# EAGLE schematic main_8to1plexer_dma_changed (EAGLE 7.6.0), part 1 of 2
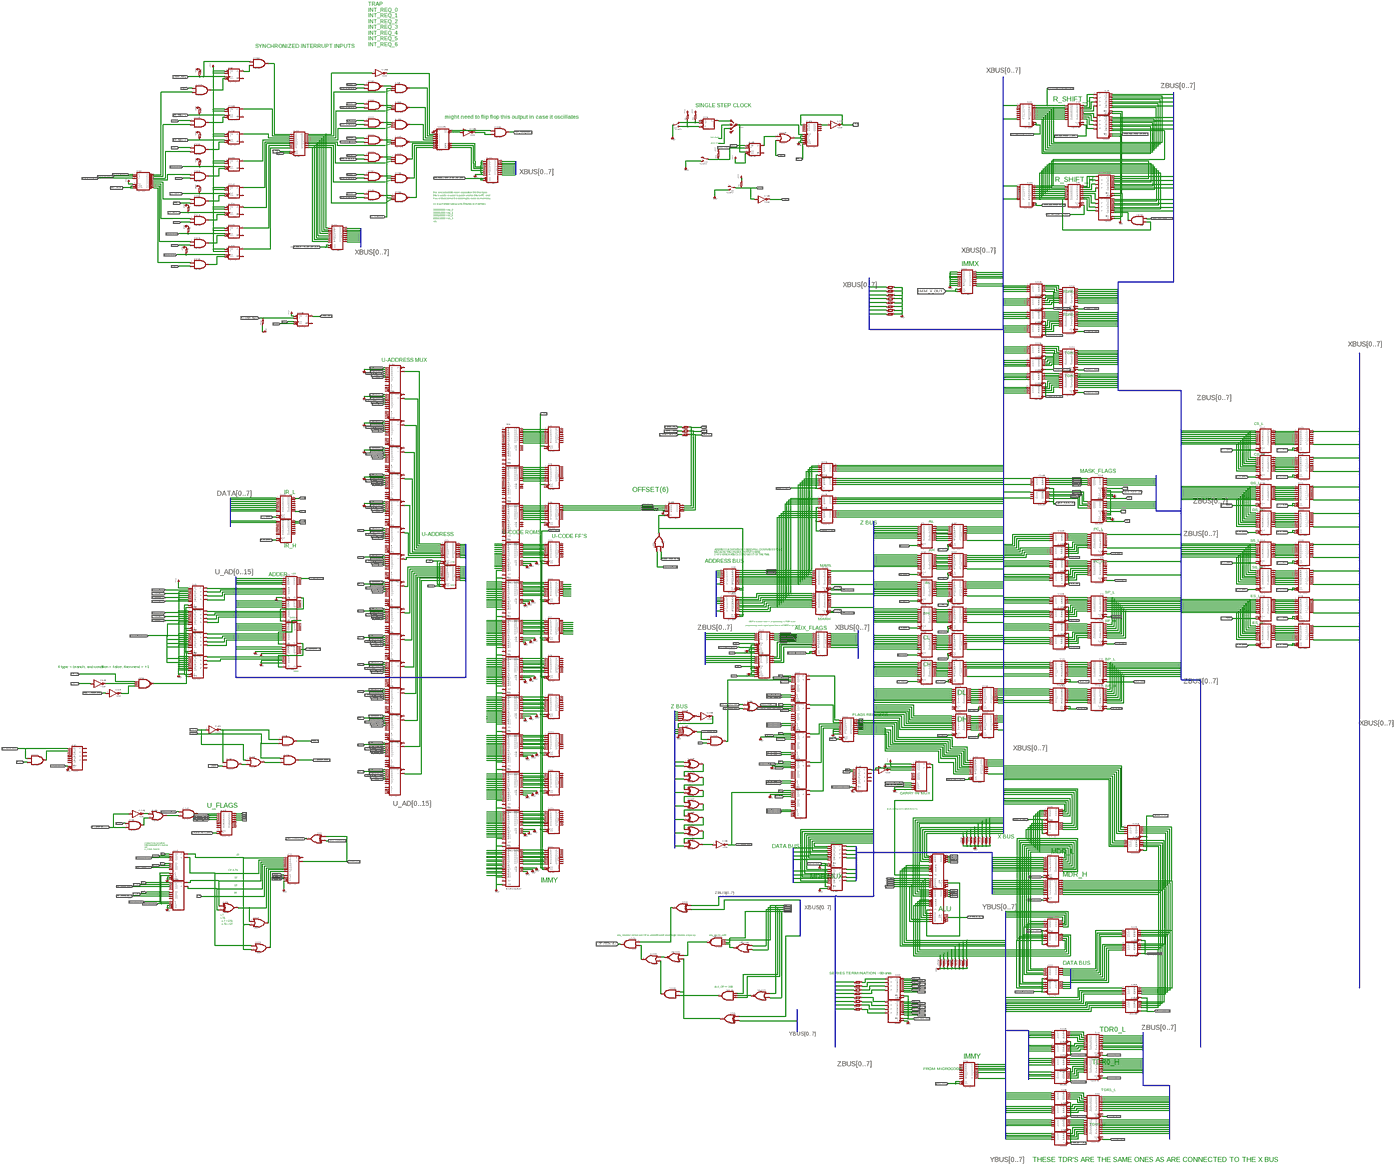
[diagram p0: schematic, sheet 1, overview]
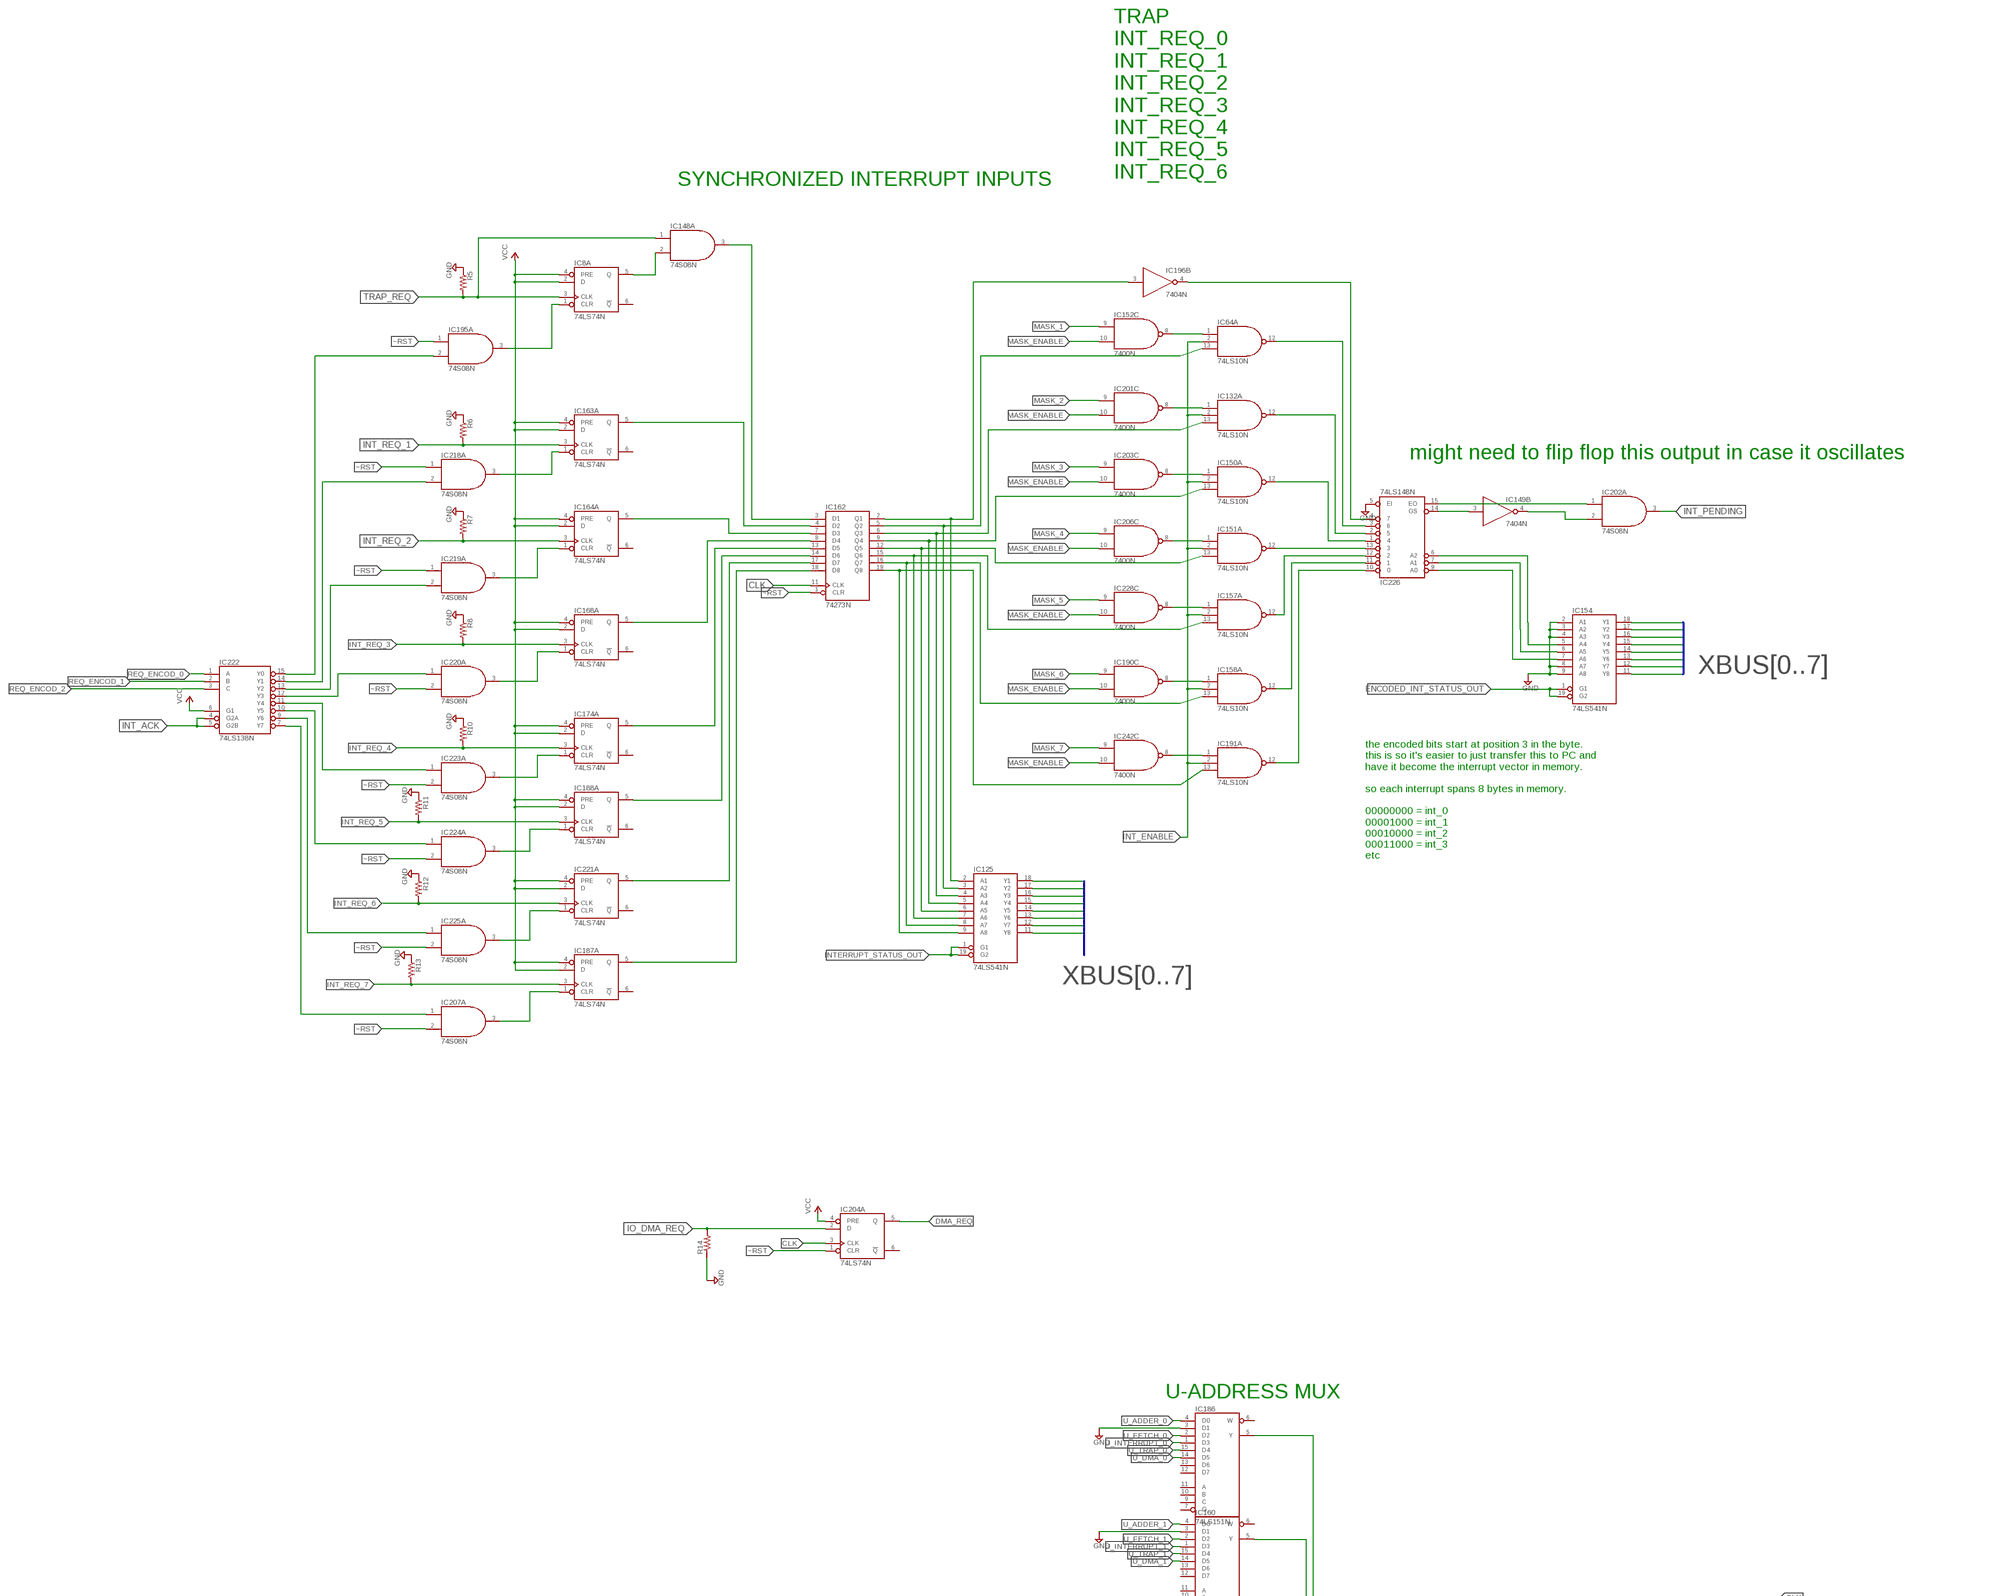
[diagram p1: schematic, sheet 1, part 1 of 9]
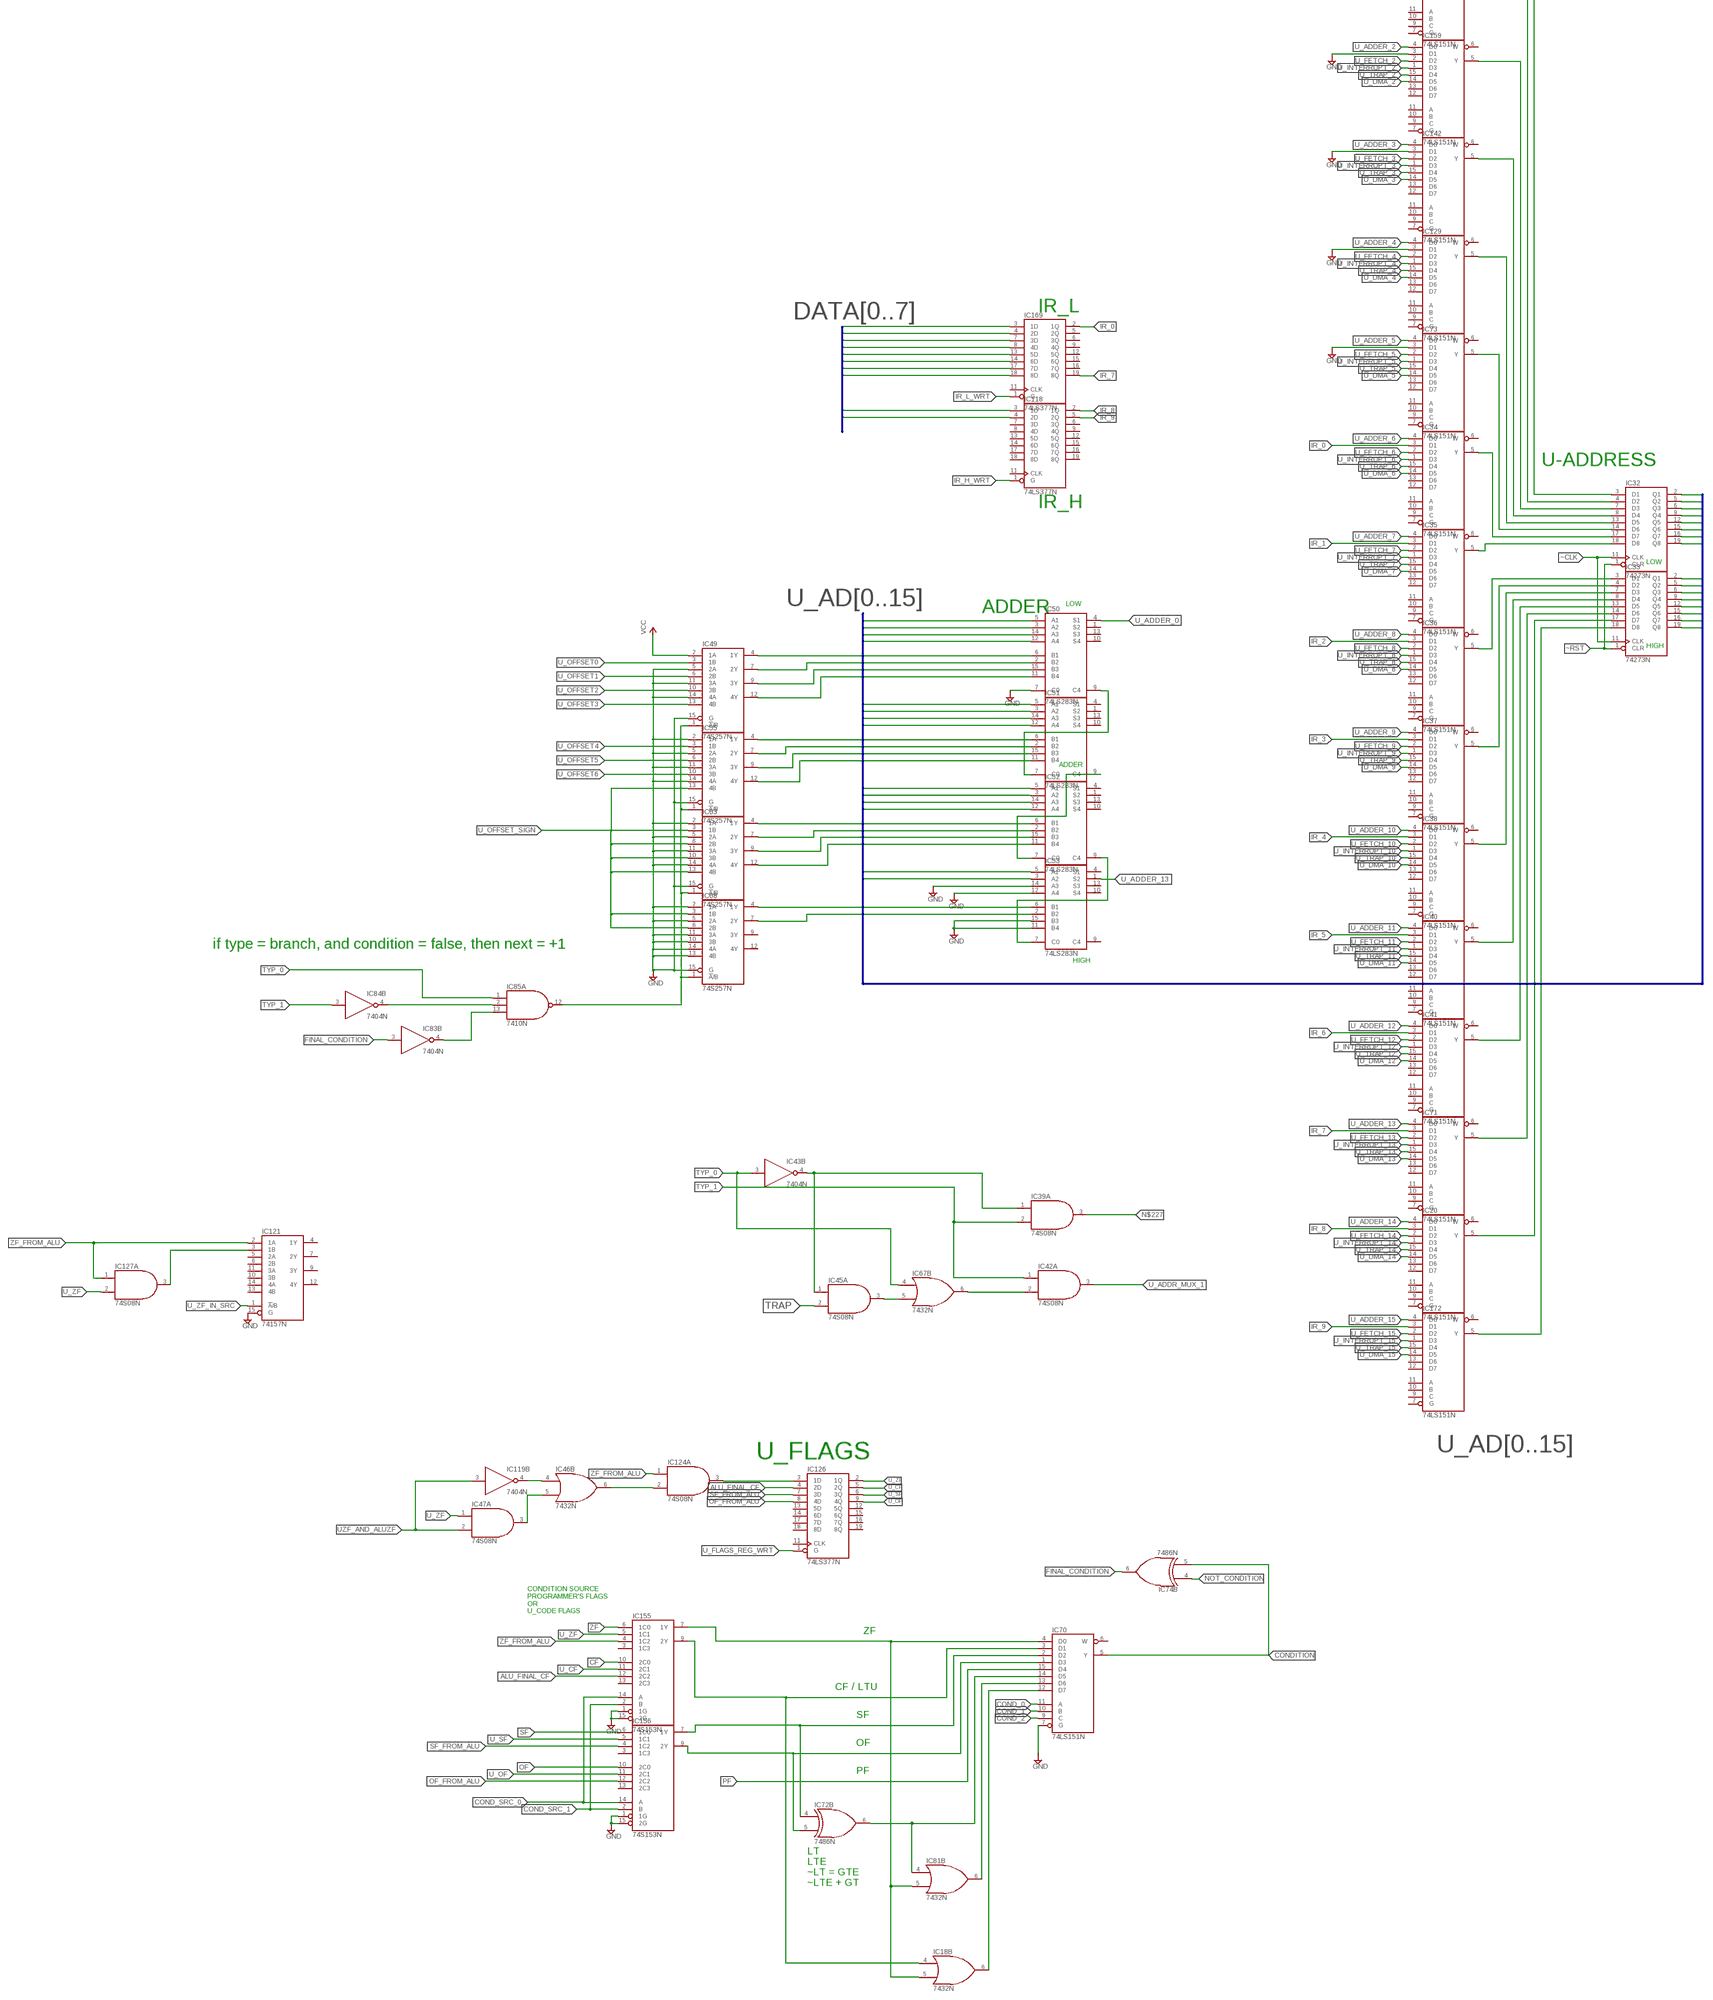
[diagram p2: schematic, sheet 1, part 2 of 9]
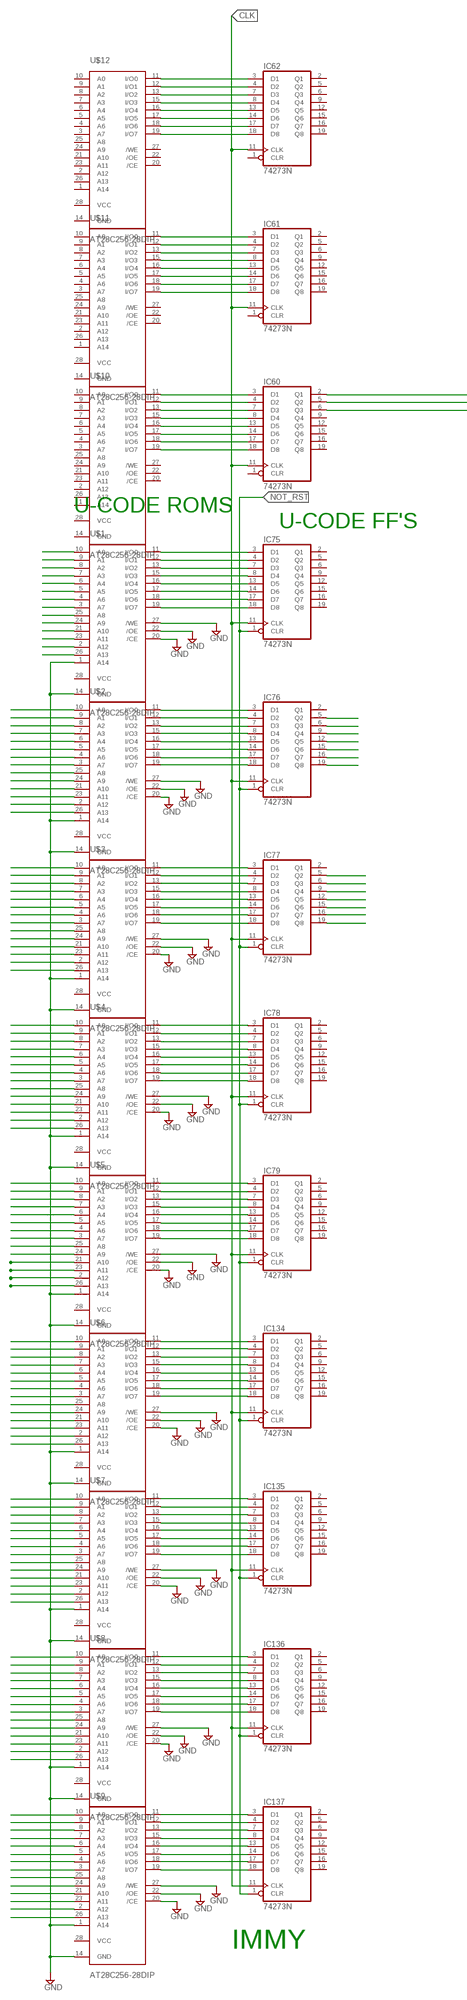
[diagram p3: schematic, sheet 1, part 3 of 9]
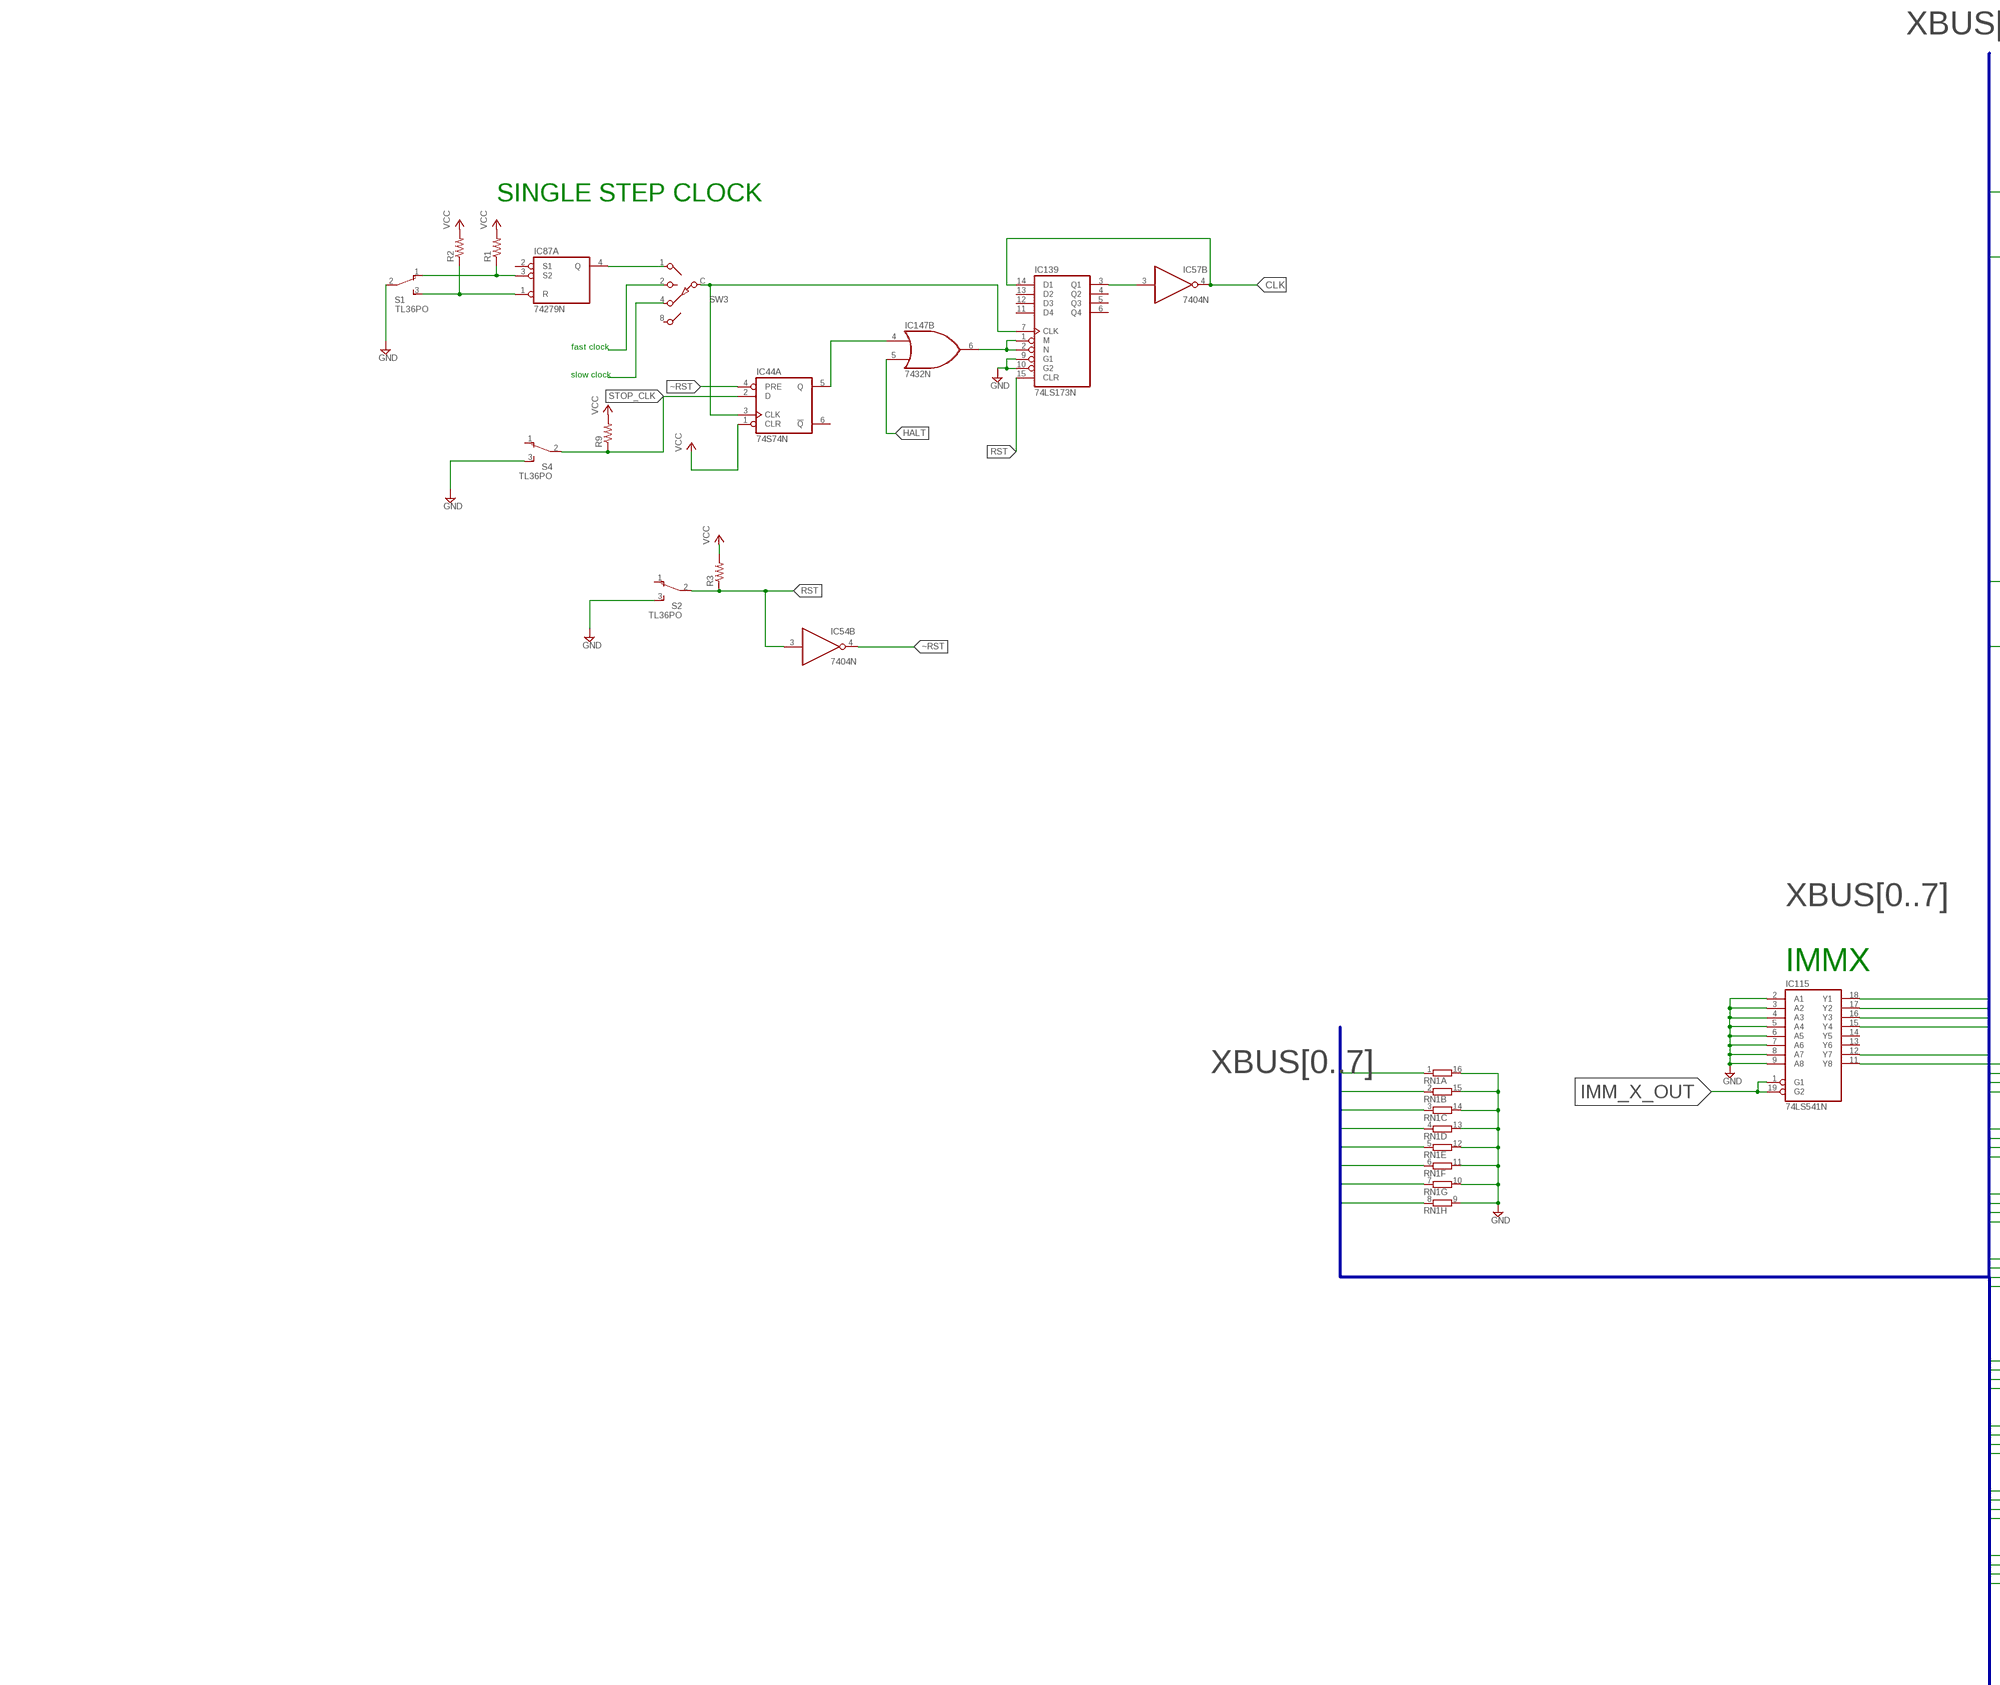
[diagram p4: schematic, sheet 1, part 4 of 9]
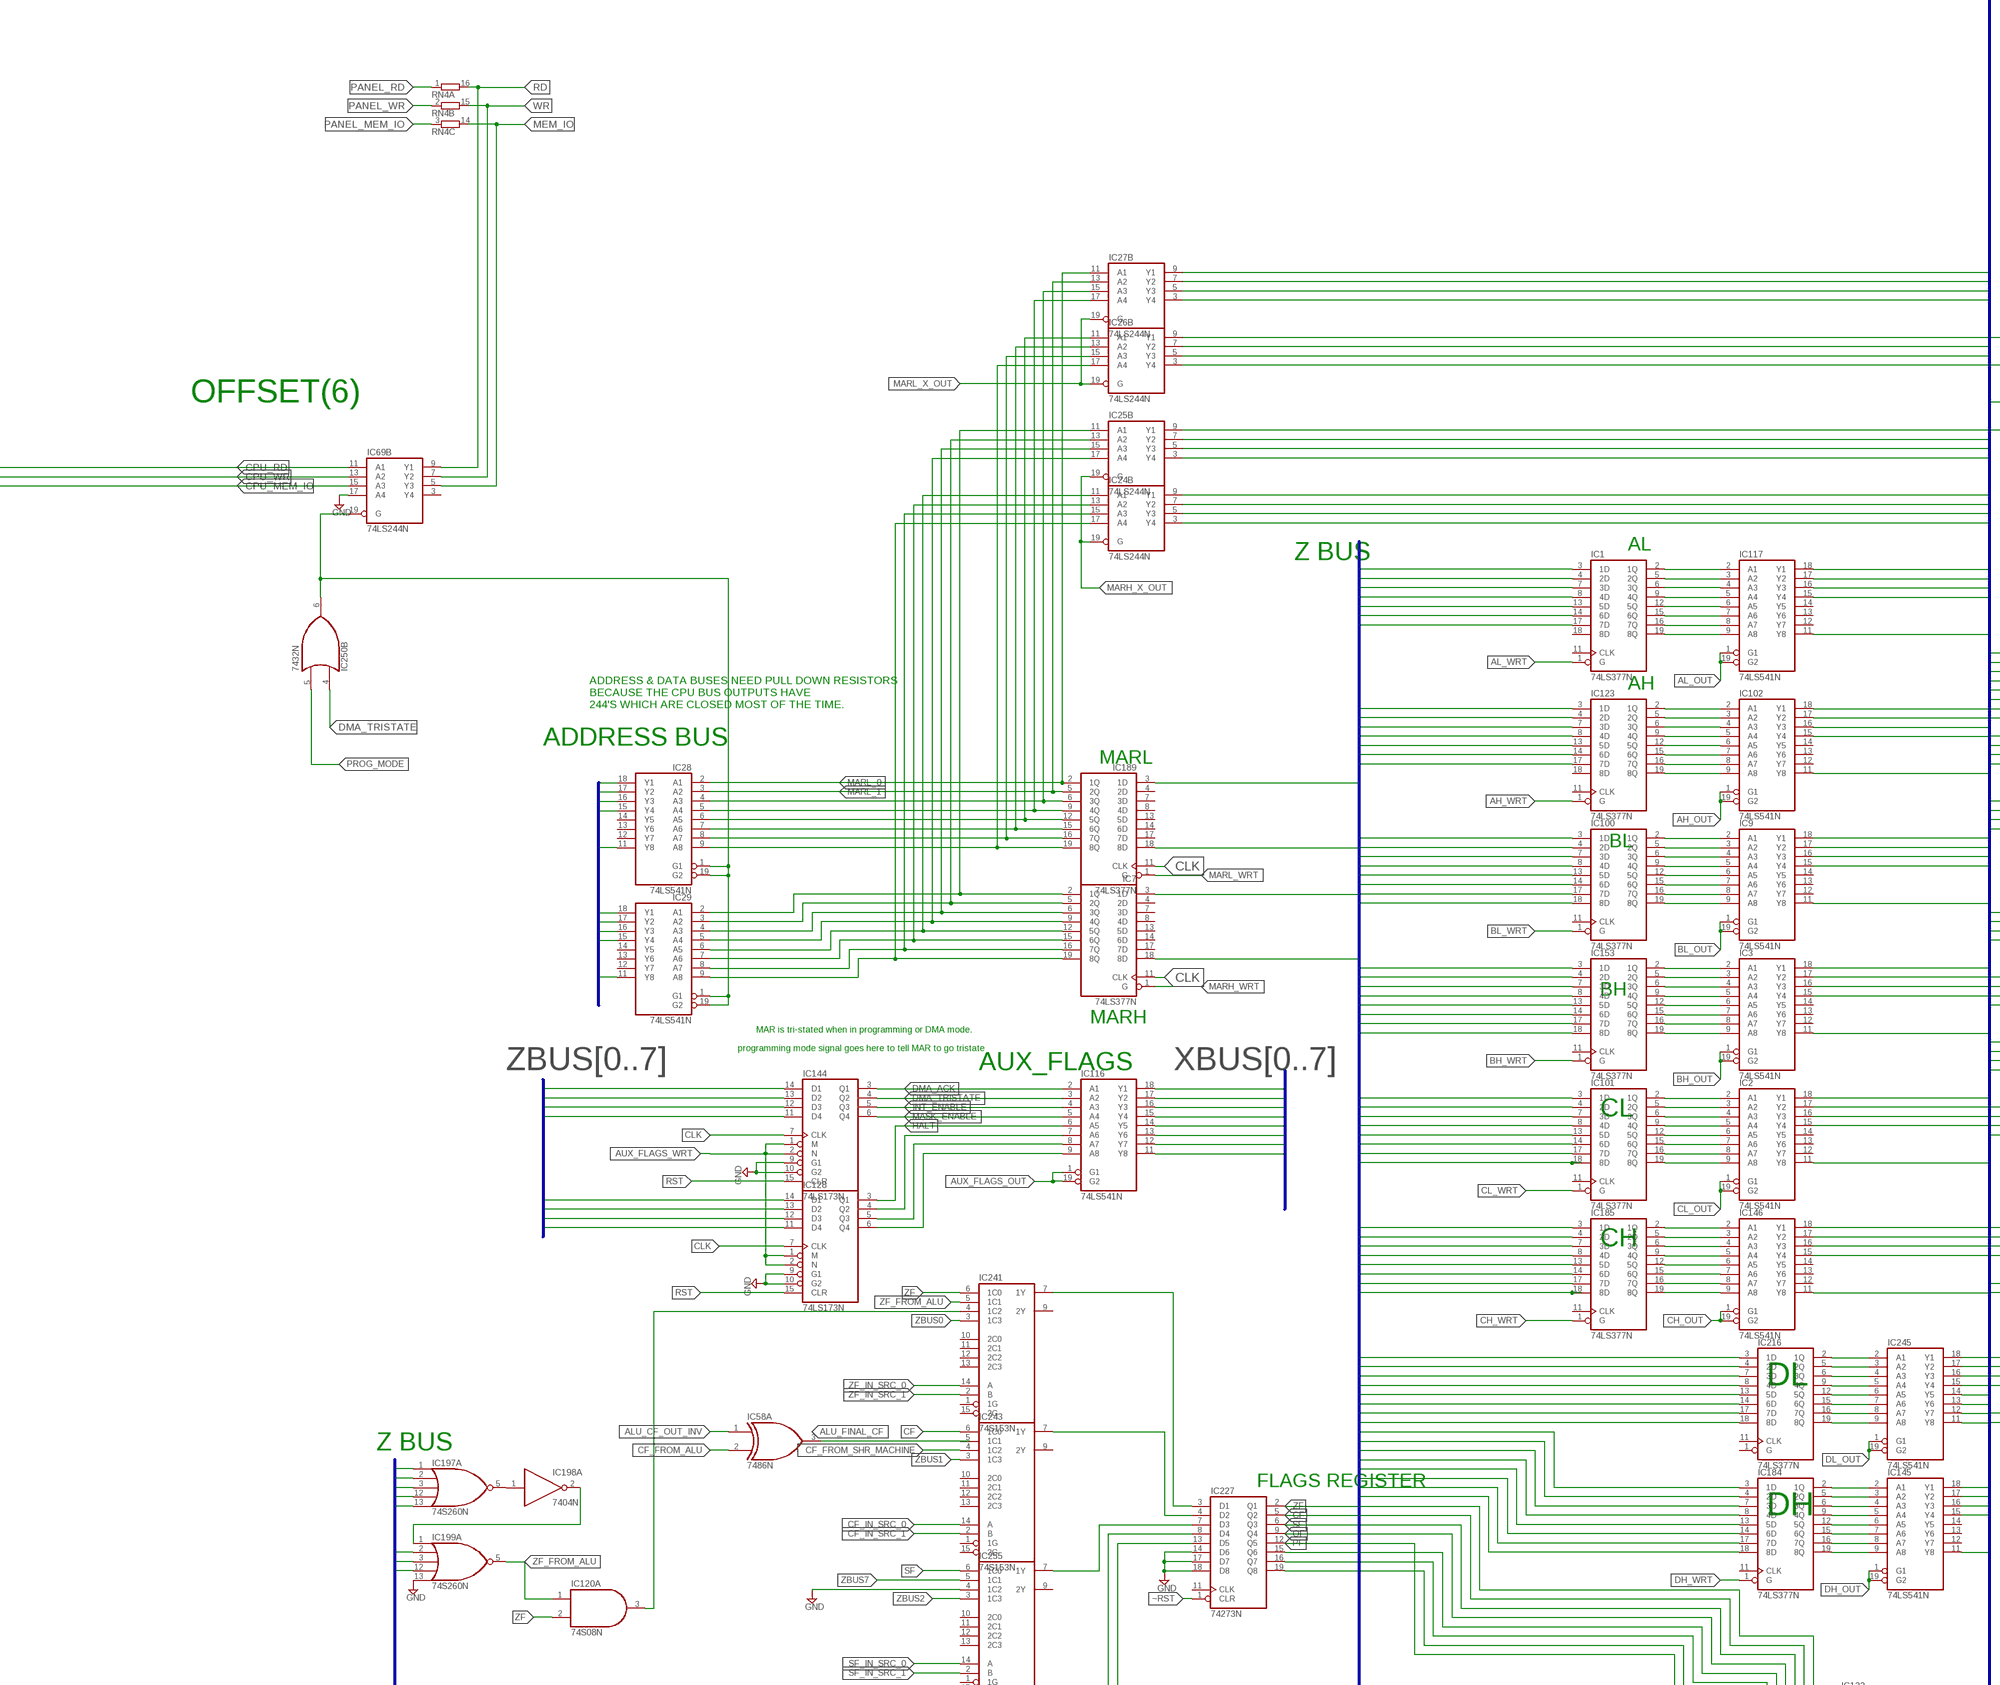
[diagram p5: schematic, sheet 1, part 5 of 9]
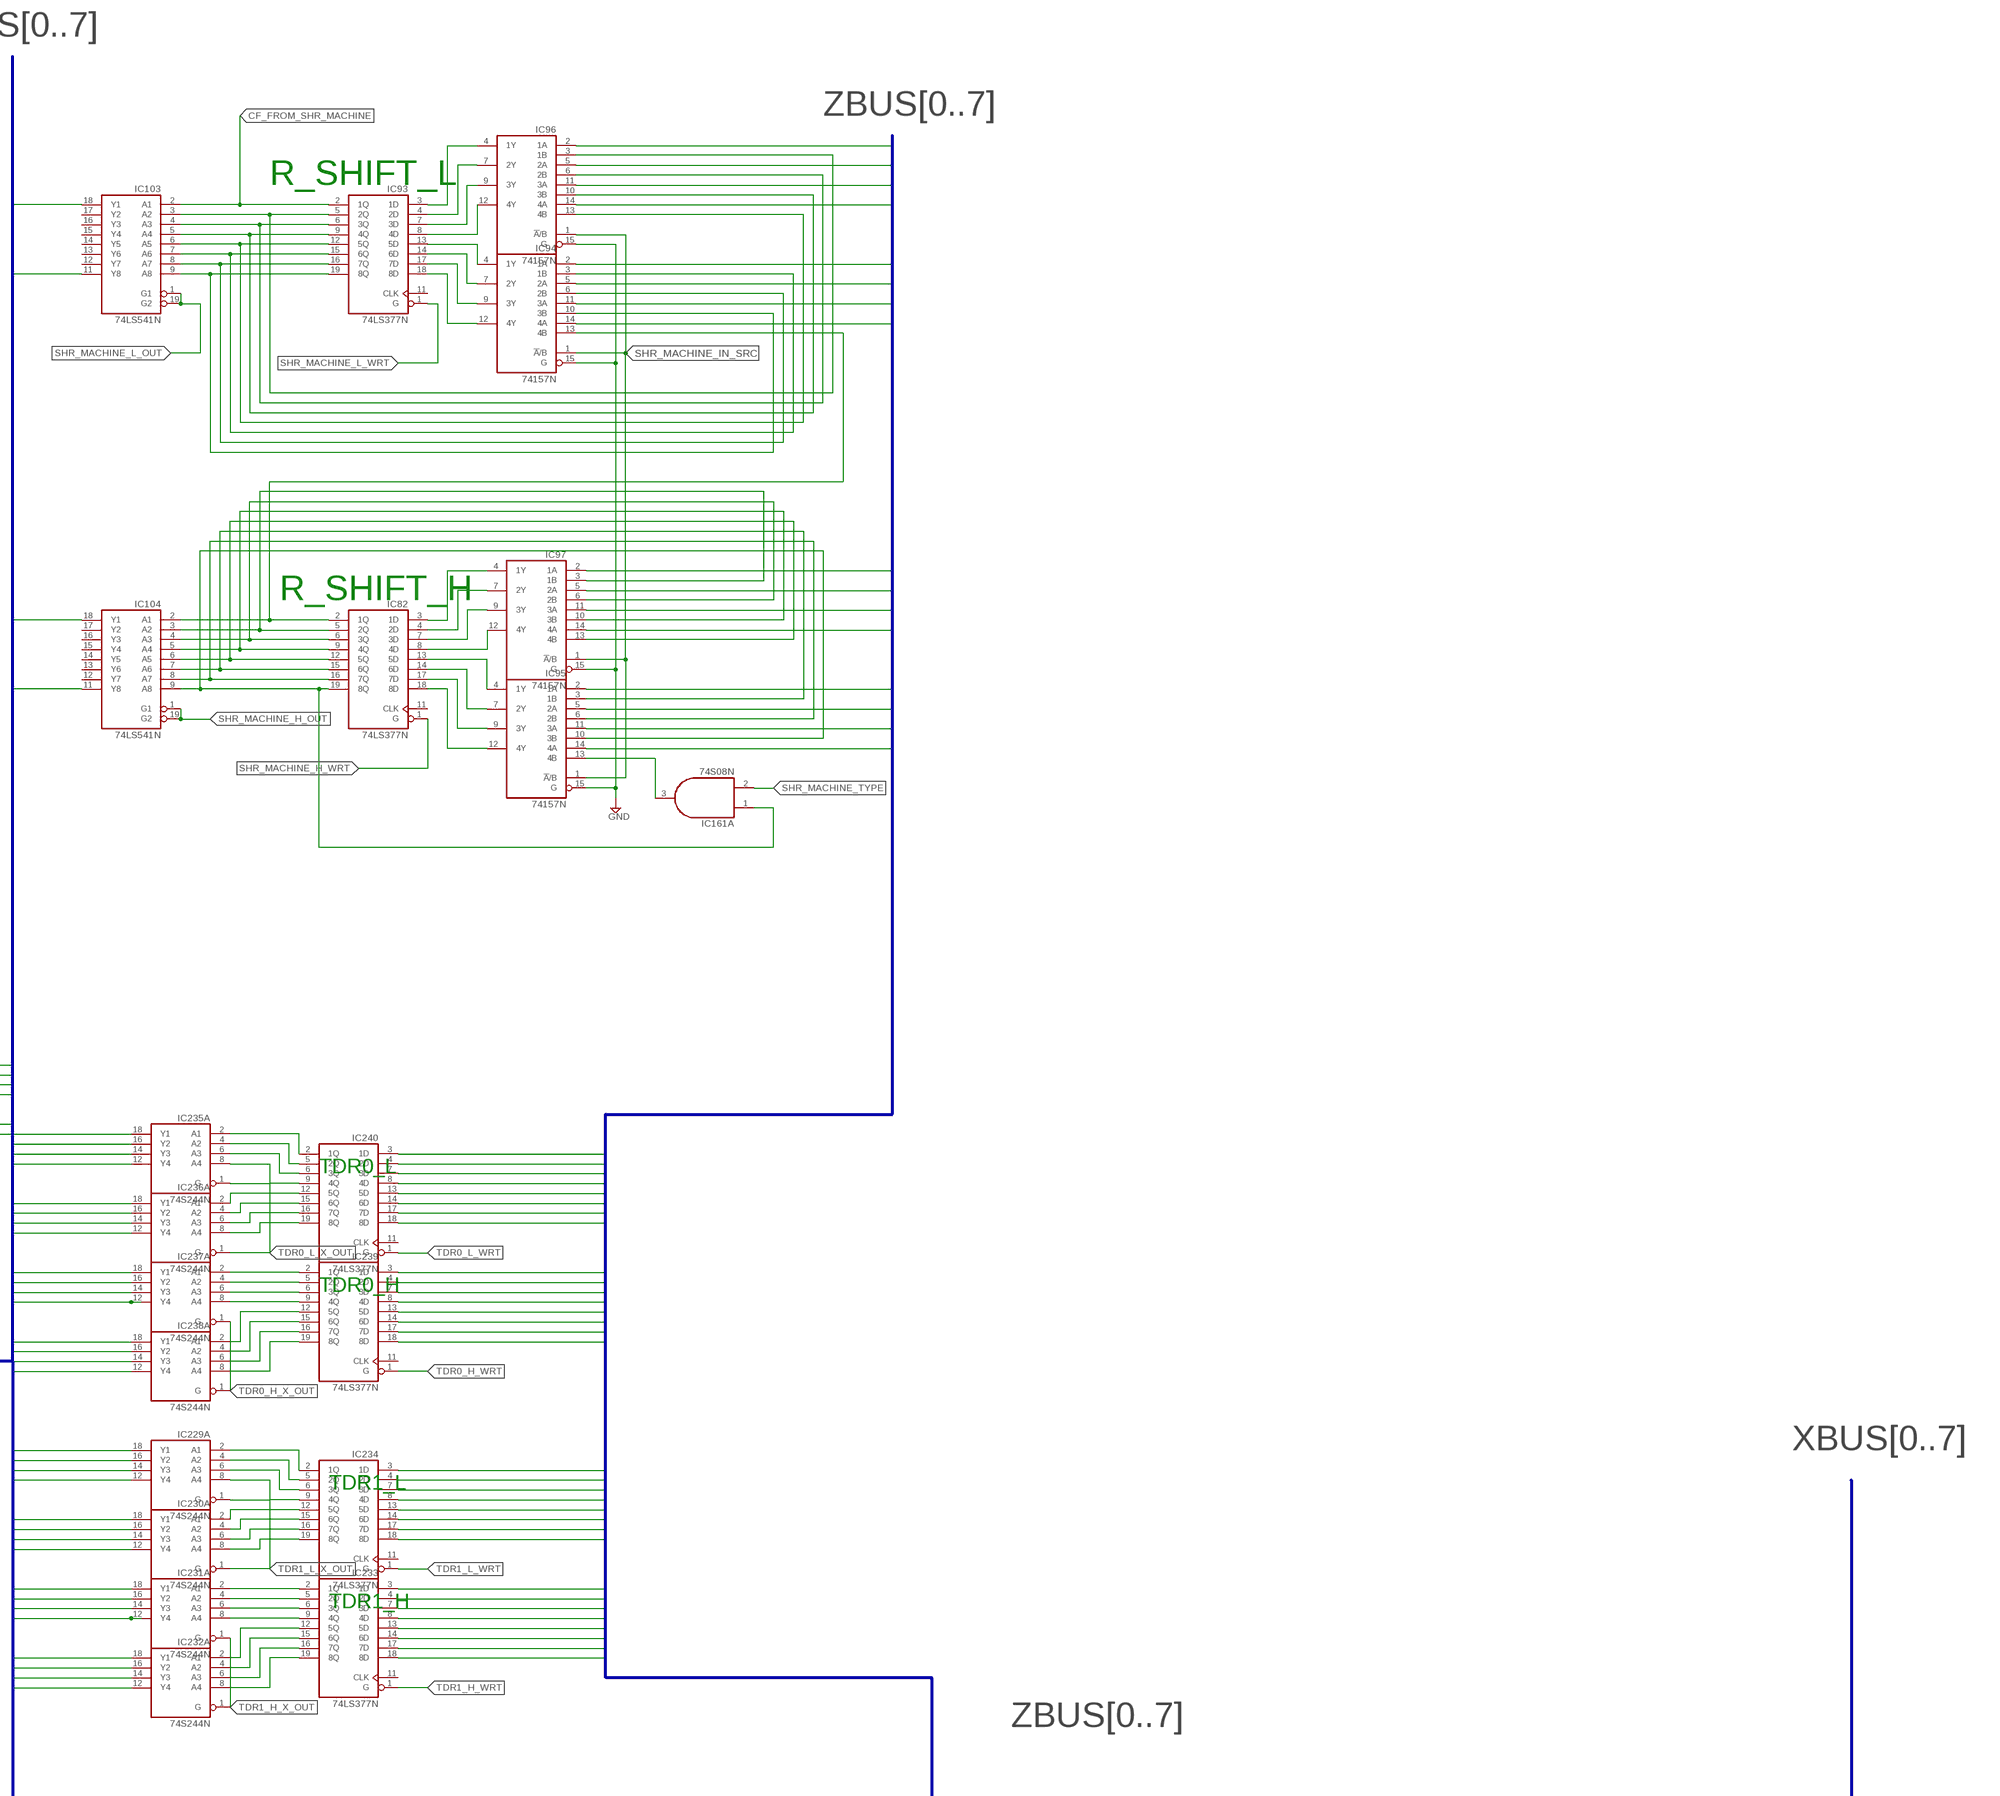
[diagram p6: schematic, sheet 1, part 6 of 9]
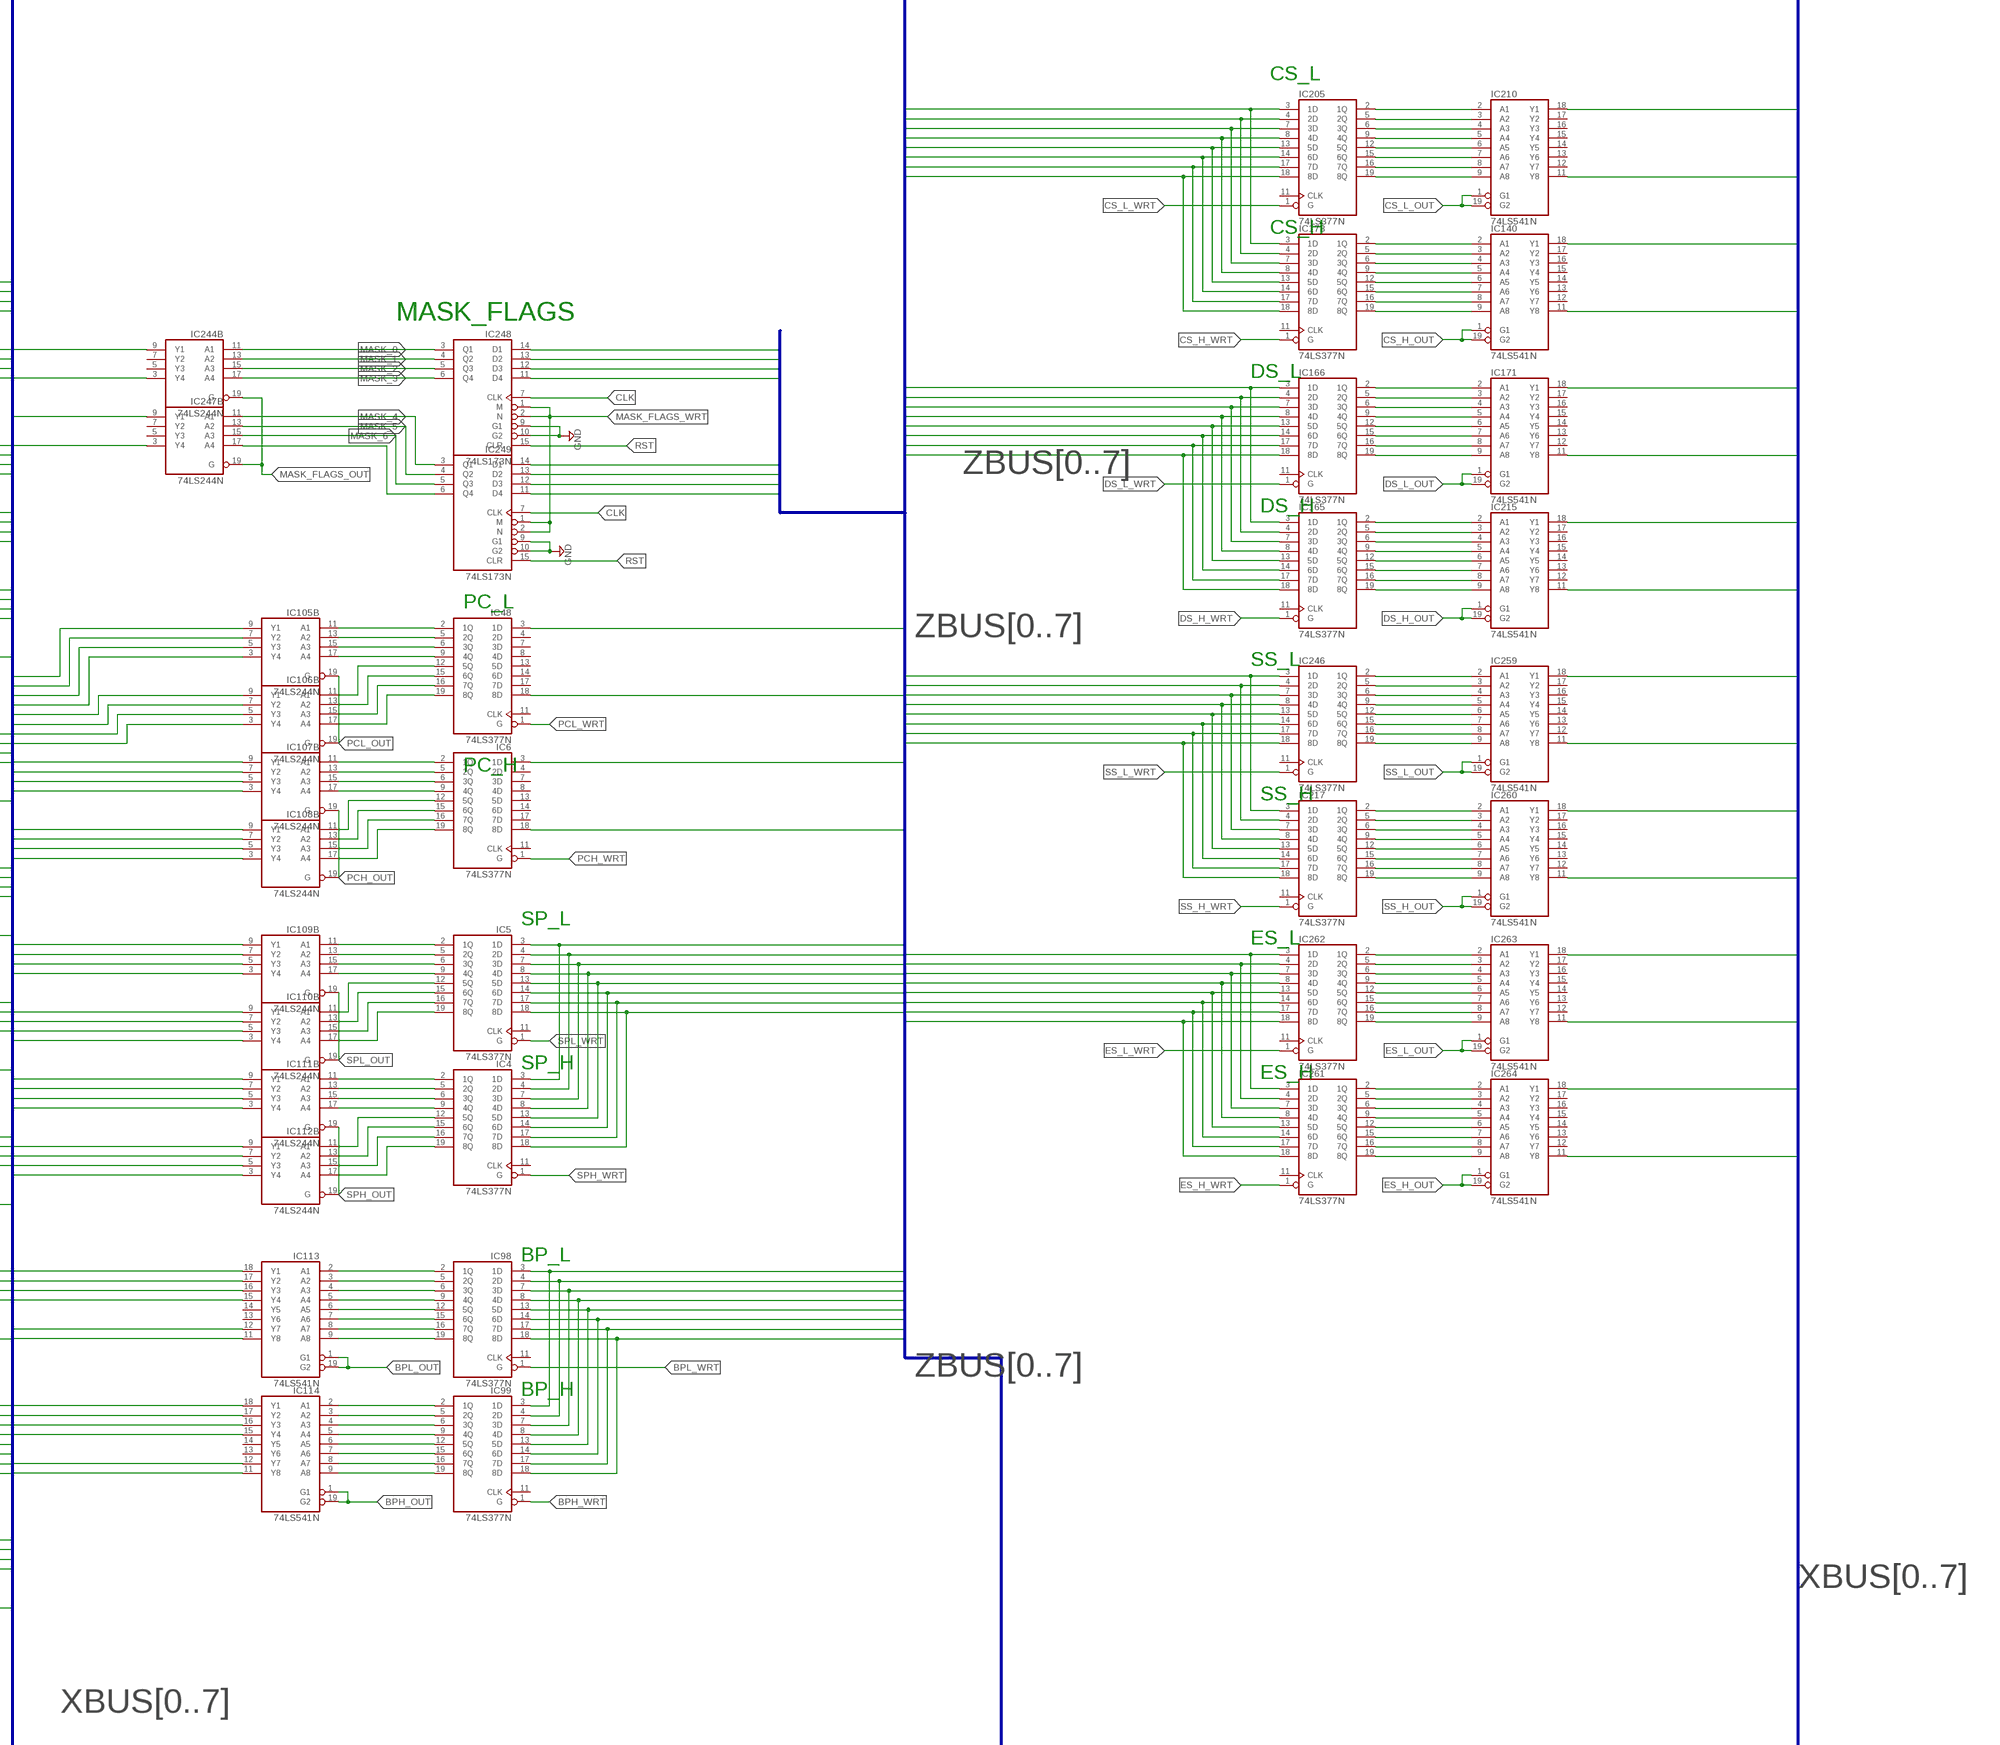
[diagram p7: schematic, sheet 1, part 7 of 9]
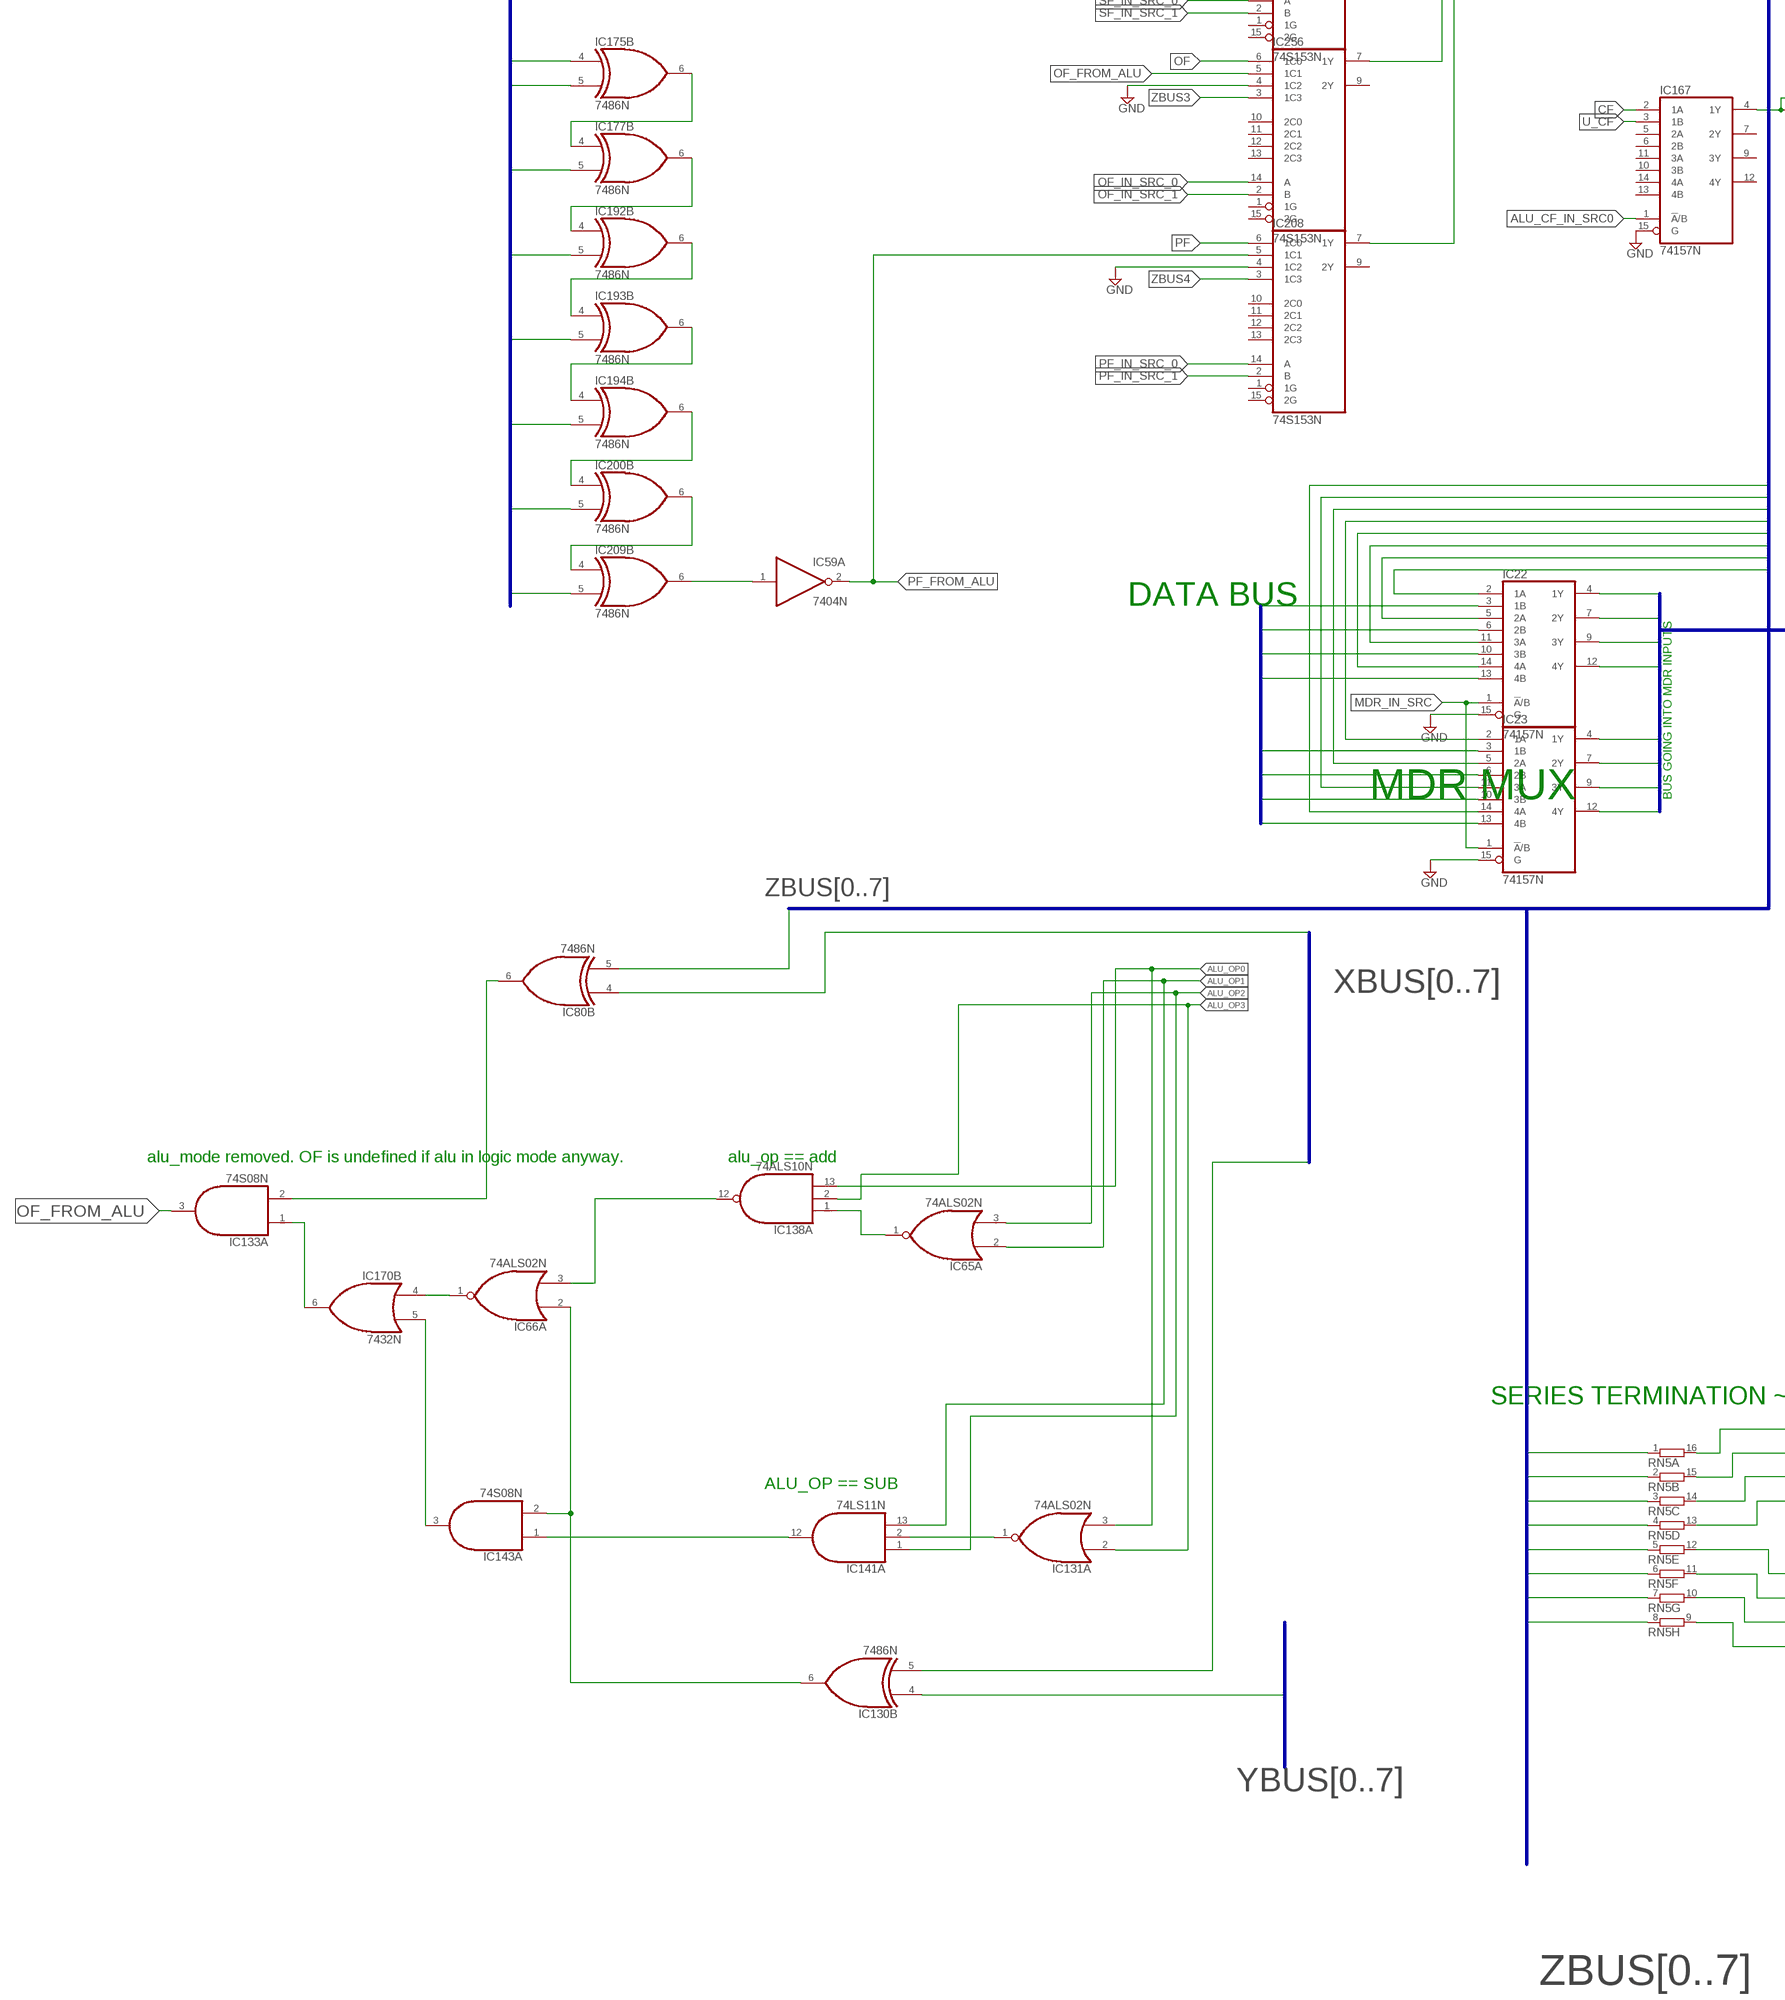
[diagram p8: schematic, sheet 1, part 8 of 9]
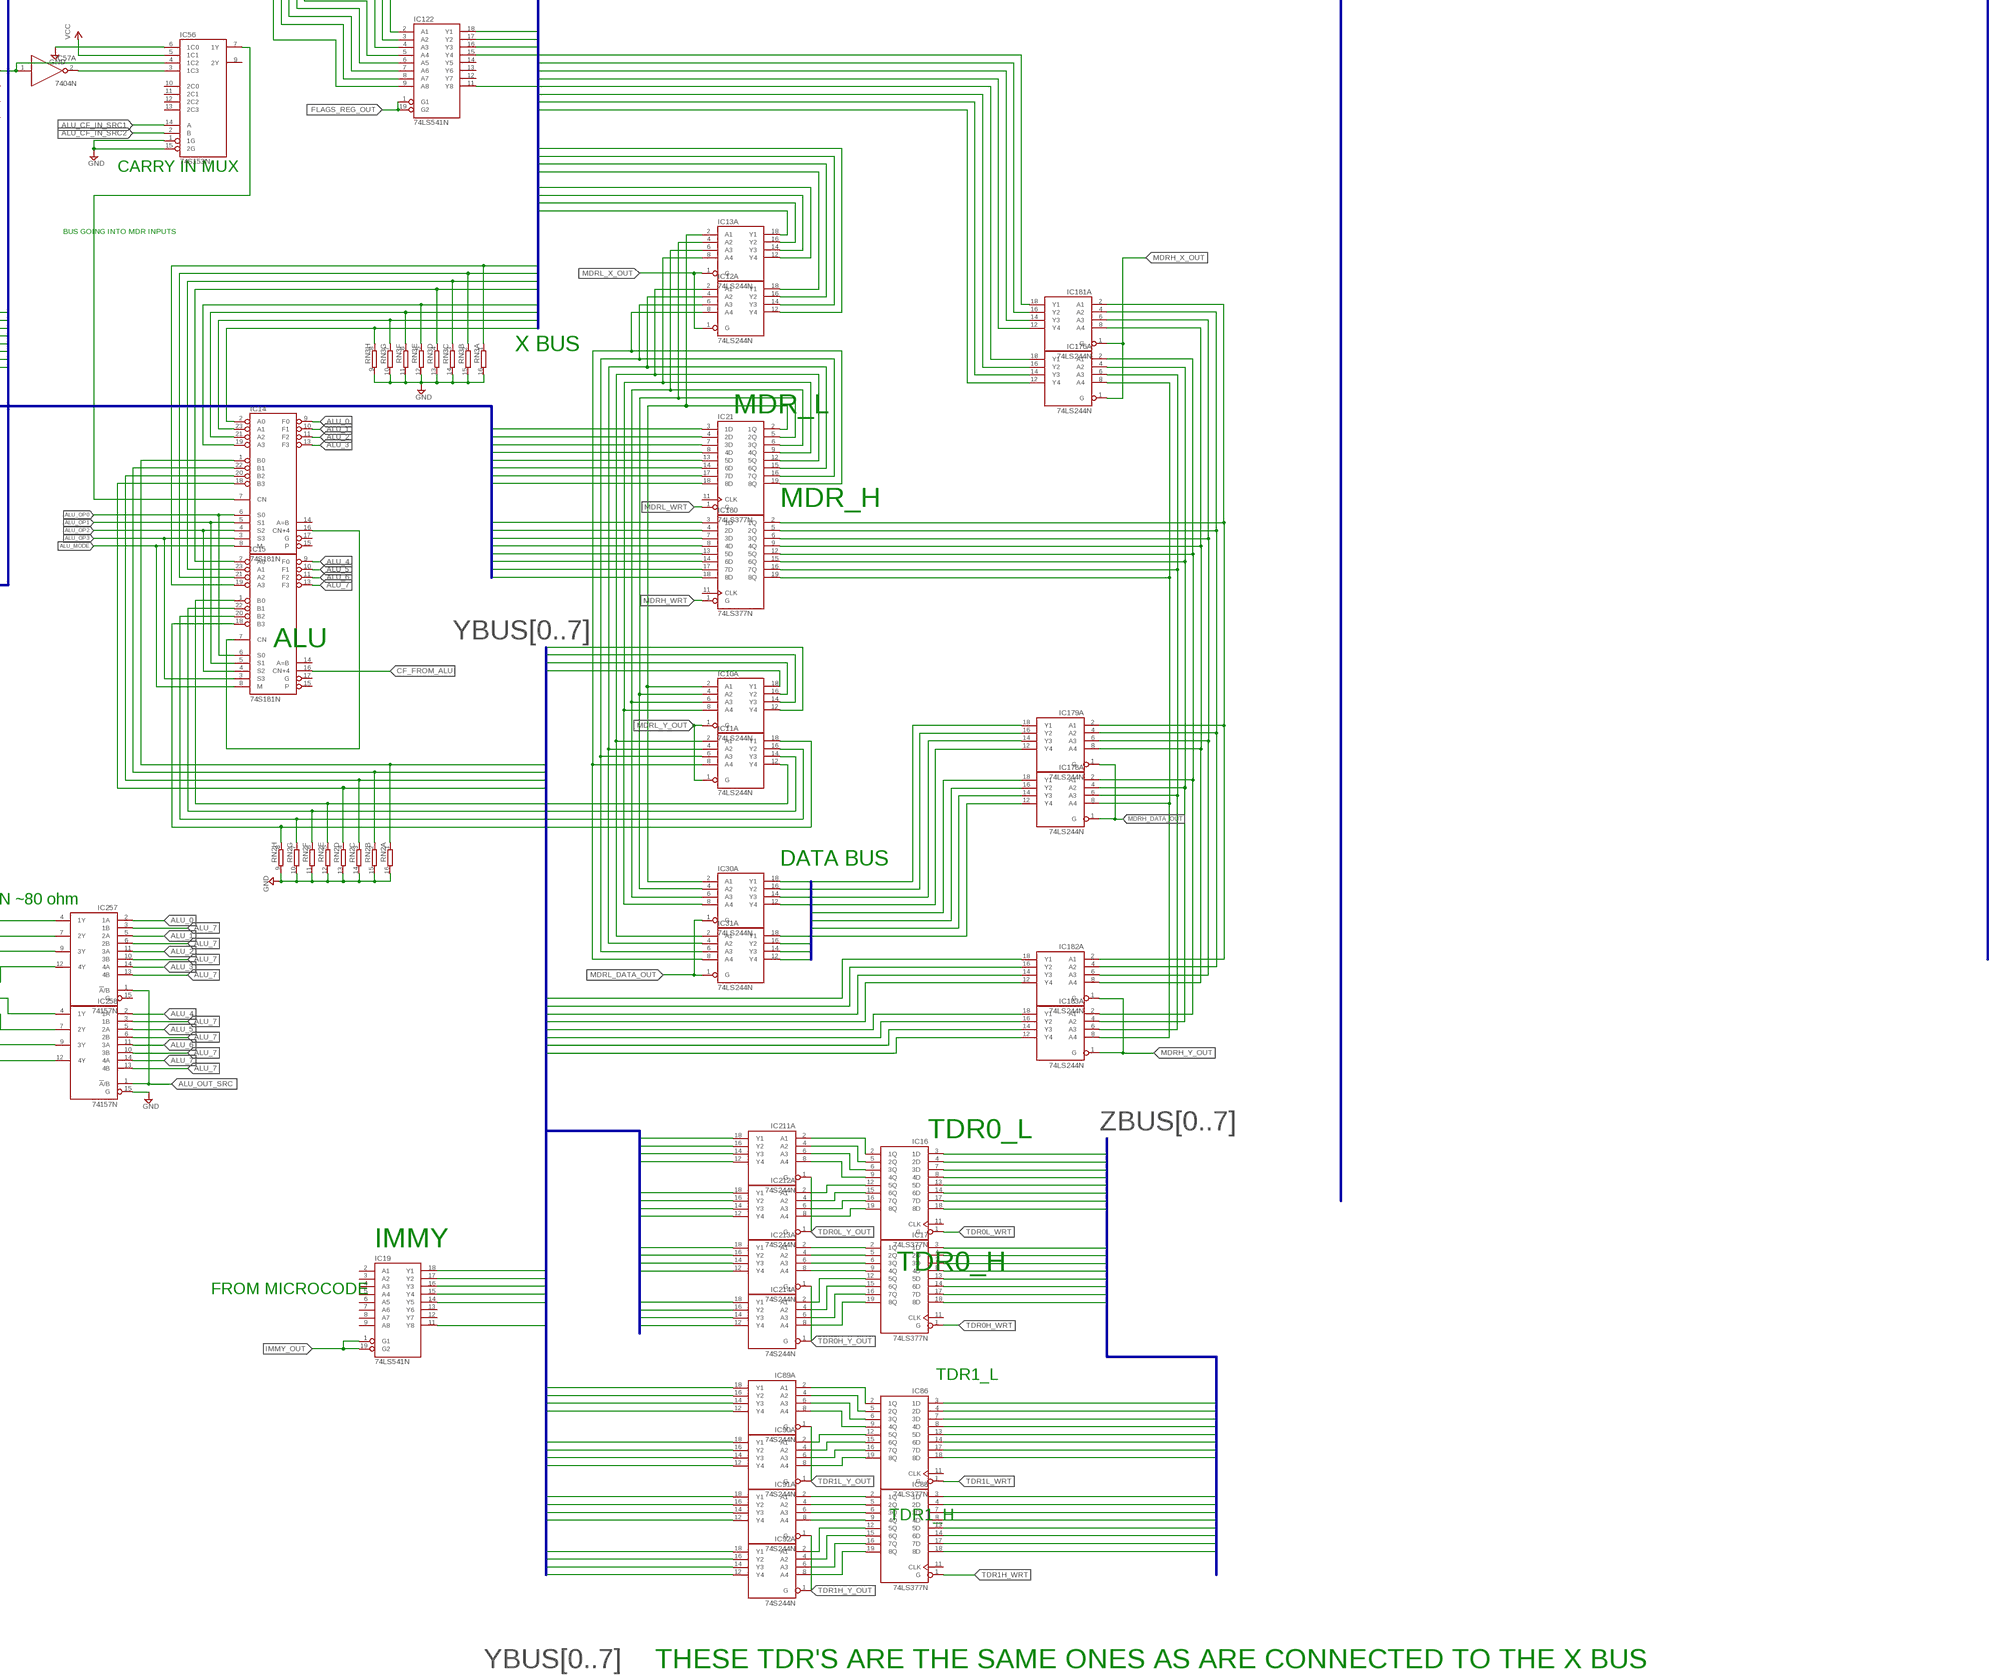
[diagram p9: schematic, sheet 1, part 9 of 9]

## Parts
IC1  74LS377N  [DIL20]
IC2  74LS541N  [DIL20]
IC3  74LS541N  [DIL20]
IC4  74LS377N  [DIL20]
IC5  74LS377N  [DIL20]
IC6  74LS377N  [DIL20]
IC7  74LS377N  [DIL20]
IC8  74LS74N  [DIL14]
IC9  74LS541N  [DIL20]
IC10  74LS244N  [DIL20]
IC11  74LS244N  [DIL20]
IC12  74LS244N  [DIL20]
IC13  74LS244N  [DIL20]
IC14  74S181N  [DIL24-6]
IC15  74S181N  [DIL24-6]
IC16  74LS377N  [DIL20]
IC17  74LS377N  [DIL20]
IC18  7432N  [DIL14]
IC19  74LS541N  [DIL20]
IC20  74LS151N  [DIL16]
IC21  74LS377N  [DIL20]
IC22  74157N  [DIL16]
IC23  74157N  [DIL16]
IC24  74LS244N  [DIL20]
IC25  74LS244N  [DIL20]
IC26  74LS244N  [DIL20]
IC27  74LS244N  [DIL20]
IC28  74LS541N  [DIL20]
IC29  74LS541N  [DIL20]
IC30  74LS244N  [DIL20]
IC31  74LS244N  [DIL20]
IC32  74273N  [DIL20]
IC33  74273N  [DIL20]
IC34  74LS151N  [DIL16]
IC35  74LS151N  [DIL16]
IC36  74LS151N  [DIL16]
IC37  74LS151N  [DIL16]
IC38  74LS151N  [DIL16]
IC39  74S08N  [DIL14]
IC40  74LS151N  [DIL16]
IC41  74LS151N  [DIL16]
IC42  74S08N  [DIL14]
IC43  7404N  [DIL14]
IC44  74S74N  [DIL14]
IC45  74S08N  [DIL14]
IC46  7432N  [DIL14]
IC47  74S08N  [DIL14]
IC48  74LS377N  [DIL20]
IC49  74S257N  [DIL16]
IC50  74LS283N  [DIL16]
IC51  74LS283N  [DIL16]
IC52  74LS283N  [DIL16]
IC53  74LS283N  [DIL16]
IC54  7404N  [DIL14]
IC55  74S257N  [DIL16]
IC56  74S153N  [DIL16]
IC57  7404N  [DIL14]
IC58  7486N  [DIL14]
IC59  7404N  [DIL14]
IC60  74273N  [DIL20]
IC61  74273N  [DIL20]
IC62  74273N  [DIL20]
IC63  74S257N  [DIL16]
IC64  74LS10N  [DIL14]
IC65  74ALS02N  [DIL14]
IC66  74ALS02N  [DIL14]
IC67  7432N  [DIL14]
IC68  74S257N  [DIL16]
IC69  74LS244N  [DIL20]
IC70  74LS151N  [DIL16]
IC71  74LS151N  [DIL16]
IC72  7486N  [DIL14]
IC73  74LS151N  [DIL16]
IC74  7486N  [DIL14]
IC75  74273N  [DIL20]
IC76  74273N  [DIL20]
IC77  74273N  [DIL20]
IC78  74273N  [DIL20]
IC79  74273N  [DIL20]
IC80  7486N  [DIL14]
IC81  7432N  [DIL14]
IC82  74LS377N  [DIL20]
IC83  7404N  [DIL14]
IC84  7404N  [DIL14]
IC85  7410N  [DIL14]
IC86  74LS377N  [DIL20]
IC87  74279N  [DIL16]
IC88  74LS377N  [DIL20]
IC89  74S244N  [DIL20]
IC90  74S244N  [DIL20]
IC91  74S244N  [DIL20]
IC92  74S244N  [DIL20]
IC93  74LS377N  [DIL20]
IC94  74157N  [DIL16]
IC95  74157N  [DIL16]
IC96  74157N  [DIL16]
IC97  74157N  [DIL16]
IC98  74LS377N  [DIL20]
IC99  74LS377N  [DIL20]
IC100  74LS377N  [DIL20]
IC101  74LS377N  [DIL20]
IC102  74LS541N  [DIL20]
IC103  74LS541N  [DIL20]
IC104  74LS541N  [DIL20]
IC105  74LS244N  [DIL20]
IC106  74LS244N  [DIL20]
IC107  74LS244N  [DIL20]
IC108  74LS244N  [DIL20]
IC109  74LS244N  [DIL20]
IC110  74LS244N  [DIL20]
IC111  74LS244N  [DIL20]
IC112  74LS244N  [DIL20]
IC113  74LS541N  [DIL20]
IC114  74LS541N  [DIL20]
IC115  74LS541N  [DIL20]
IC116  74LS541N  [DIL20]
IC117  74LS541N  [DIL20]
IC118  74LS377N  [DIL20]
IC119  7404N  [DIL14]
IC120  74S08N  [DIL14]
IC121  74157N  [DIL16]
IC122  74LS541N  [DIL20]
IC123  74LS377N  [DIL20]
IC124  74S08N  [DIL14]
IC125  74LS541N  [DIL20]
IC126  74LS377N  [DIL20]
IC127  74S08N  [DIL14]
IC128  74LS173N  [DIL16]
IC129  74LS151N  [DIL16]
IC130  7486N  [DIL14]
IC131  74ALS02N  [DIL14]
IC132  74LS10N  [DIL14]
IC133  74S08N  [DIL14]
IC134  74273N  [DIL20]
IC135  74273N  [DIL20]
IC136  74273N  [DIL20]
IC137  74273N  [DIL20]
IC138  74ALS10N  [DIL14]
IC139  74LS173N  [DIL16]
IC140  74LS541N  [DIL20]
IC141  74LS11N  [DIL14]
IC142  74LS151N  [DIL16]
IC143  74S08N  [DIL14]
IC144  74LS173N  [DIL16]
IC145  74LS541N  [DIL20]
IC146  74LS541N  [DIL20]
IC147  7432N  [DIL14]
IC148  74S08N  [DIL14]
IC149  7404N  [DIL14]
IC150  74LS10N  [DIL14]
IC151  74LS10N  [DIL14]
IC152  7400N  [DIL14]
IC153  74LS377N  [DIL20]
IC154  74LS541N  [DIL20]
IC155  74S153N  [DIL16]
IC156  74S153N  [DIL16]
IC157  74LS10N  [DIL14]
IC158  74LS10N  [DIL14]
IC159  74LS151N  [DIL16]
IC160  74LS151N  [DIL16]
IC161  74S08N  [DIL14]
IC162  74273N  [DIL20]
IC163  74LS74N  [DIL14]
IC164  74LS74N  [DIL14]
IC165  74LS377N  [DIL20]
IC166  74LS377N  [DIL20]
IC167  74157N  [DIL16]
IC168  74LS74N  [DIL14]
IC169  74LS377N  [DIL20]
IC170  7432N  [DIL14]
IC171  74LS541N  [DIL20]
IC172  74LS151N  [DIL16]
IC173  74LS377N  [DIL20]
IC174  74LS74N  [DIL14]
IC175  7486N  [DIL14]
IC176  74LS244N  [DIL20]
IC177  7486N  [DIL14]
IC178  74LS244N  [DIL20]
IC179  74LS244N  [DIL20]
IC180  74LS377N  [DIL20]
IC181  74LS244N  [DIL20]
IC182  74LS244N  [DIL20]
IC183  74LS244N  [DIL20]
IC184  74LS377N  [DIL20]
IC185  74LS377N  [DIL20]
IC186  74LS151N  [DIL16]
IC187  74LS74N  [DIL14]
IC188  74LS74N  [DIL14]
IC189  74LS377N  [DIL20]
IC190  7400N  [DIL14]
IC191  74LS10N  [DIL14]
IC192  7486N  [DIL14]
IC193  7486N  [DIL14]
IC194  7486N  [DIL14]
IC195  74S08N  [DIL14]
IC196  7404N  [DIL14]
IC197  74S260N  [DIL14]
IC198  7404N  [DIL14]
IC199  74S260N  [DIL14]
IC200  7486N  [DIL14]
IC201  7400N  [DIL14]
IC202  74S08N  [DIL14]
IC203  7400N  [DIL14]
IC204  74LS74N  [DIL14]
IC205  74LS377N  [DIL20]
IC206  7400N  [DIL14]
IC207  74S08N  [DIL14]
IC208  74S153N  [DIL16]
IC209  7486N  [DIL14]
IC210  74LS541N  [DIL20]
IC211  74S244N  [DIL20]
IC212  74S244N  [DIL20]
IC213  74S244N  [DIL20]
IC214  74S244N  [DIL20]
IC215  74LS541N  [DIL20]
IC216  74LS377N  [DIL20]
IC217  74LS377N  [DIL20]
IC218  74S08N  [DIL14]
IC219  74S08N  [DIL14]
IC220  74S08N  [DIL14]
IC221  74LS74N  [DIL14]
IC222  74LS138N  [DIL16]
IC223  74S08N  [DIL14]
IC224  74S08N  [DIL14]
IC225  74S08N  [DIL14]
IC226  74LS148N  [DIL16]
IC227  74273N  [DIL20]
IC228  7400N  [DIL14]
IC229  74S244N  [DIL20]
IC230  74S244N  [DIL20]
IC231  74S244N  [DIL20]
IC232  74S244N  [DIL20]
IC233  74LS377N  [DIL20]
IC234  74LS377N  [DIL20]
IC235  74S244N  [DIL20]
IC236  74S244N  [DIL20]
IC237  74S244N  [DIL20]
IC238  74S244N  [DIL20]
IC239  74LS377N  [DIL20]
IC240  74LS377N  [DIL20]
IC241  74S153N  [DIL16]
IC242  7400N  [DIL14]
IC243  74S153N  [DIL16]
IC244  74LS244N  [DIL20]
IC245  74LS541N  [DIL20]
IC246  74LS377N  [DIL20]
IC247  74LS244N  [DIL20]
IC248  74LS173N  [DIL16]
IC249  74LS173N  [DIL16]
IC250  7432N  [DIL14]
IC255  74S153N  [DIL16]
IC256  74S153N  [DIL16]
IC257  74157N  [DIL16]
IC258  74157N  [DIL16]
IC259  74LS541N  [DIL20]
IC260  74LS541N  [DIL20]
IC261  74LS377N  [DIL20]
IC262  74LS377N  [DIL20]
IC263  74LS541N  [DIL20]
IC264  74LS541N  [DIL20]
R1  R-US_0204/2V  [0204V]
R2  R-US_0204/2V  [0204V]
R3  R-US_0204/2V  [0204V]
R5  R-US_0204/7  [0204/7]
R6  R-US_0204/7  [0204/7]
R7  R-US_0204/7  [0204/7]
R8  R-US_0204/7  [0204/7]
R9  R-US_0204/2V  [0204V]
R10  R-US_0204/7  [0204/7]
R11  R-US_0204/7  [0204/7]
R12  R-US_0204/7  [0204/7]
R13  R-US_0204/7  [0204/7]
R14  R-US_0204/7  [0204/7]
RN1  8R-N  [DIL16]
RN2  8R-N  [DIL16]
RN3  8R-N  [DIL16]
RN4  8R-N  [DIL16]
RN5  8R-N  [DIL16]
S1  TL36PO  [TL3XPO]
S2  TL36PO  [TL3XPO]
S4  TL36PO  [TL3XPO]
SW3  SW-C10  [SW-C10]
U$1  AT28C256-28DIP  [DIL28-6]
U$2  AT28C256-28DIP  [DIL28-6]
U$3  AT28C256-28DIP  [DIL28-6]
U$4  AT28C256-28DIP  [DIL28-6]
U$5  AT28C256-28DIP  [DIL28-6]
U$6  AT28C256-28DIP  [DIL28-6]
U$7  AT28C256-28DIP  [DIL28-6]
U$8  AT28C256-28DIP  [DIL28-6]
U$9  AT28C256-28DIP  [DIL28-6]
U$10  AT28C256-28DIP  [DIL28-6]
U$11  AT28C256-28DIP  [DIL28-6]
U$12  AT28C256-28DIP  [DIL28-6]

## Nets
45435: IC18.5(B:I1) IC70.4(D0) IC81.5(B:I1) IC155.7(1Y)
345345: IC70.2(D2) IC72.4(B:I0) IC156.7(1Y)
634354: IC18.4(B:I0) IC70.3(D1) IC155.9(2Y)
654654: IC122.7(A6) IC227.16(Q7)
4654654: IC70.1(D3) IC72.5(B:I1) IC156.9(2Y)
5434534: IC122.6(A5) IC227.15(Q6)
AD0: IC28.18(Y1)
AD1: IC28.17(Y2)
AD2: IC28.16(Y3)
AD3: IC28.15(Y4)
AD7: IC28.11(Y8)
AD8: IC29.18(Y1)
AD9: IC29.17(Y2)
AD10: IC29.16(Y3)
AD11: IC29.15(Y4)
AD15: IC29.11(Y8)
AH_OUT: IC102.1(G1) IC102.19(G2)
AH_WRT: IC123.1(G)
AL_OUT: IC117.1(G1) IC117.19(G2)
AL_WRT: IC1.1(G)
ALU_0: IC14.9(F0) IC257.2(1A)
ALU_1: IC14.10(F1) IC257.5(2A)
ALU_2: IC14.11(F2) IC257.11(3A)
ALU_3: IC14.13(F3) IC257.14(4A)
ALU_4: IC15.9(F0) IC258.2(1A)
ALU_5: IC15.10(F1) IC258.5(2A)
ALU_6: IC15.11(F2) IC258.11(3A)
ALU_7: IC15.13(F3) IC257.3(1B) IC257.6(2B) IC257.10(3B) IC257.13(4B) IC258.3(1B) IC258.6(2B) IC258.10(3B) IC258.13(4B) IC258.14(4A)
ALU_CF_IN_SRC0: IC167.1(!A!/B)
ALU_CF_IN_SRC1: IC56.14(A)
ALU_CF_IN_SRC2: IC56.2(B)
ALU_CF_OUT_INV: IC58.1(A:I0)
ALU_FINAL_CF: IC58.3(A:O) IC126.4(2D) IC155.12(2C2) IC243.5(1C1)
ALU_MODE: IC14.8(M) IC15.8(M)
ALU_OP0: IC14.6(S0) IC15.6(S0) IC131.3(A:I1) IC138.13(A:I2)
ALU_OP1: IC14.5(S1) IC15.5(S1) IC65.2(A:I0) IC141.13(A:I2)
ALU_OP2: IC14.4(S2) IC15.4(S2) IC65.3(A:I1) IC141.1(A:I0)
ALU_OP3: IC14.3(S3) IC15.3(S3) IC131.2(A:I0) IC138.2(A:I1)
ALU_OUT_SRC: IC257.1(!A!/B) IC258.1(!A!/B)
AUX_FLAGS_OUT: IC116.1(G1) IC116.19(G2)
AUX_FLAGS_WRT: IC128.1(M) IC128.2(N) IC144.1(M) IC144.2(N)
BH_OUT: IC3.1(G1) IC3.19(G2)
BH_WRT: IC153.1(G)
BL_OUT: IC9.1(G1) IC9.19(G2)
BL_WRT: IC100.1(G)
BPH_OUT: IC114.1(G1)
BPH_WRT: IC99.1(G)
BPL_OUT: IC113.1(G1)
BPL_WRT: IC98.1(G)
CF: IC122.3(A2) IC155.10(2C0) IC167.2(1A) IC227.5(Q2) IC243.6(1C0)
CF_FROM_ALU: IC15.16(CN+4) IC58.2(A:I1)
CF_FROM_SHR_MACHINE: IC93.2(1Q) IC103.2(A1) IC243.4(1C2)
CF_IN_SRC_0: IC243.14(A)
CF_IN_SRC_1: IC243.2(B)
CH_OUT: IC146.1(G1) IC146.19(G2)
CH_WRT: IC185.1(G)
CL_OUT: IC2.1(G1) IC2.19(G2)
CL_WRT: IC101.1(G)
CLK: IC7.11(CLK) IC57.4(B:O) IC60.11(CLK) IC61.11(CLK) IC62.11(CLK) IC75.11(CLK) IC76.11(CLK) IC77.11(CLK) IC78.11(CLK) IC79.11(CLK) IC128.7(CLK) IC134.11(CLK) IC135.11(CLK) IC136.11(CLK) IC137.11(CLK) IC139.14(D1) IC144.7(CLK) IC162.11(CLK) IC189.11(CLK) IC204.3(A:CLK) IC248.7(CLK) IC249.7(CLK)
COND_0: IC70.11(A)
COND_1: IC70.10(B)
COND_2: IC70.9(C)
COND_SRC_0: IC155.14(A) IC156.14(A)
COND_SRC_1: IC155.2(B) IC156.2(B)
CONDITION: IC70.5(Y) IC74.5(B:I1)
CPU_MEM_IO: IC60.6(Q3) IC69.15(B:A3)
CPU_RD: IC60.2(Q1) IC69.11(B:A1)
CPU_WR: IC60.5(Q2) IC69.13(B:A2)
CS_H_OUT: IC140.1(G1) IC140.19(G2)
CS_H_WRT: IC173.1(G)
CS_L_OUT: IC210.1(G1) IC210.19(G2)
CS_L_WRT: IC205.1(G)
DATA0: IC118.3(1D) IC169.3(1D) IC179.18(A:Y1)
DATA1: IC118.4(2D) IC169.4(2D) IC179.16(A:Y2)
DATA2: IC169.7(3D) IC179.14(A:Y3)
DATA3: IC169.8(4D) IC179.12(A:Y4)
DATA4: IC169.13(5D) IC178.18(A:Y1)
DATA5: IC169.14(6D) IC178.16(A:Y2)
DATA6: IC169.17(7D) IC178.14(A:Y3)
DATA7: IC169.18(8D) IC178.12(A:Y4)
DH_OUT: IC145.1(G1) IC145.19(G2)
DH_WRT: IC184.1(G)
DL_OUT: IC245.1(G1) IC245.19(G2)
DMA_ACK: IC116.2(A1) IC144.3(Q1)
DMA_REQ: IC204.5(A:Q)
DMA_TRISTATE: IC28.1(G1) IC28.19(G2) IC29.1(G1) IC29.19(G2) IC69.19(B:G) IC116.3(A2) IC144.4(Q2) IC250.4(B:I0) IC250.6(B:O)
DS_H_OUT: IC215.1(G1) IC215.19(G2)
DS_H_WRT: IC165.1(G)
DS_L_OUT: IC171.1(G1) IC171.19(G2)
DS_L_WRT: IC166.1(G)
ENCODED_INT_STATUS_OUT: IC154.1(G1) IC154.19(G2)
ES_H_OUT: IC264.1(G1) IC264.19(G2)
ES_H_WRT: IC261.1(G)
ES_L_OUT: IC263.1(G1) IC263.19(G2)
ES_L_WRT: IC262.1(G)
FINAL_CONDITION: IC74.6(B:O) IC83.3(B:I)
FLAGS_REG_OUT: IC122.1(G1) IC122.19(G2)
GND: IC22.15(G) IC23.15(G) IC49.5(2A) IC49.11(3A) IC49.14(4A) IC49.15(G) IC50.7(C0) IC53.11(B4) IC53.12(A4) IC53.14(A3) IC53.15(B3) IC55.2(1A) IC55.5(2A) IC55.11(3A) IC55.14(4A) IC55.15(G) IC56.1(1G) IC56.6(1C0) IC56.15(2G) IC63.2(1A) IC63.5(2A) IC63.11(3A) IC63.14(4A) IC63.15(G) IC68.2(1A) IC68.5(2A) IC68.10(3B) IC68.11(3A) IC68.13(4B) IC68.14(4A) IC68.15(G) IC69.17(B:A4) IC70.7(G) IC73.3(D1) IC94.15(G) IC95.15(G) IC96.15(G) IC97.15(G) IC115.2(A1) IC115.3(A2) IC115.4(A3) IC115.5(A4) IC115.6(A5) IC115.7(A6) IC115.8(A7) IC115.9(A8) IC121.15(G) IC128.9(G1) IC128.10(G2) IC129.3(D1) IC139.9(G1) IC139.10(G2) IC142.3(D1) IC144.9(G1) IC144.10(G2) IC154.2(A1) IC154.3(A2) IC154.4(A3) IC154.8(A7) IC154.9(A8) IC155.1(1G) IC155.15(2G) IC156.1(1G) IC156.15(2G) IC159.3(D1) IC160.3(D1) IC167.15(G) IC186.3(D1) IC199.13(A:I4) IC208.4(1C2) IC226.5(EI) IC227.14(D6) IC227.17(D7) IC227.18(D8) IC248.9(G1) IC248.10(G2) IC249.9(G1) IC249.10(G2) IC255.4(1C2) IC256.4(1C2) IC258.15(G) R5.1 R6.1 R7.1 R8.1 R10.1 R11.1 R12.1 R13.1 R14.1 RN1.9 RN1.10 RN1.11 RN1.12 RN1.13 RN1.14 RN1.15 RN1.16 RN2.9 RN2.10 RN2.11 RN2.12 RN2.13 RN2.14 RN2.15 RN2.16 RN3.9 RN3.10 RN3.11 RN3.12 RN3.13 RN3.14 RN3.15 RN3.16 S1.2(P) S2.3(S) S4.3(S) U$1.1(A14) U$1.14(GND) U$1.20(/CE) U$1.22(/OE) U$1.27(/WE) U$2.1(A14) U$2.14(GND) U$2.20(/CE) U$2.22(/OE) U$2.27(/WE) U$3.1(A14) U$3.14(GND) U$3.20(/CE) U$3.22(/OE) U$3.27(/WE) U$4.1(A14) U$4.14(GND) U$4.20(/CE) U$4.22(/OE) U$4.27(/WE) U$5.1(A14) U$5.14(GND) U$5.20(/CE) U$5.22(/OE) U$5.27(/WE) U$6.1(A14) U$6.14(GND) U$6.20(/CE) U$6.22(/OE) U$6.27(/WE) U$7.1(A14) U$7.14(GND) U$7.20(/CE) U$7.22(/OE) U$7.27(/WE) U$8.1(A14) U$8.14(GND) U$8.20(/CE) U$8.22(/OE) U$8.27(/WE) U$9.1(A14) U$9.14(GND) U$9.20(/CE) U$9.22(/OE) U$9.27(/WE)
HALT: IC116.6(A5) IC128.3(Q1) IC147.5(B:I1)
IMM_X_OUT: IC115.1(G1) IC115.19(G2)
IMMY_OUT: IC19.1(G1)
INT_ACK: IC222.4(G2A) IC222.5(G2B)
INT_ENABLE: IC64.2(A:I1) IC116.4(A3) IC132.2(A:I1) IC144.5(Q3) IC150.2(A:I1) IC151.2(A:I1) IC157.2(A:I1) IC158.2(A:I1) IC191.2(A:I1)
INT_PENDING: IC202.3(A:O)
INT_REQ_1: IC163.3(A:CLK) R6.2
INT_REQ_2: IC164.3(A:CLK) R7.2
INT_REQ_3: IC168.3(A:CLK) R8.2
INT_REQ_4: IC174.3(A:CLK) R10.2
INT_REQ_5: IC188.3(A:CLK) R11.2
INT_REQ_6: IC221.3(A:CLK) R12.2
INT_REQ_7: IC187.3(A:CLK) R13.2
INTERRUPT_STATUS_OUT: IC125.1(G1) IC125.19(G2)
IO_DMA_REQ: IC204.2(A:D) R14.2
IR_0: IC34.3(D1) IC169.2(1Q)
IR_1: IC35.3(D1)
IR_2: IC36.3(D1)
IR_3: IC37.3(D1)
IR_4: IC38.3(D1)
IR_5: IC40.3(D1)
IR_6: IC41.3(D1)
IR_7: IC71.3(D1) IC169.19(8Q)
IR_8: IC118.2(1Q)
IR_9: IC118.5(2Q)
IR_H_WRT: IC118.1(G)
IR_L_WRT: IC169.1(G)
MARH_WRT: IC7.1(G)
MARH_X_OUT: IC24.19(B:G) IC25.19(B:G)
MARL_0: IC27.11(B:A1) IC28.2(A1) IC189.2(1Q)
MARL_1: IC27.13(B:A2) IC28.3(A2) IC189.5(2Q)
MARL_WRT: IC189.1(G)
MARL_X_OUT: IC26.19(B:G) IC27.19(B:G)
MASK_0: IC244.11(B:A1) IC248.3(Q1)
MASK_1: IC152.9(C:I0) IC244.13(B:A2) IC248.4(Q2)
MASK_2: IC201.9(C:I0) IC244.15(B:A3) IC248.5(Q3)
MASK_3: IC203.9(C:I0) IC244.17(B:A4) IC248.6(Q4)
MASK_4: IC206.9(C:I0) IC247.11(B:A1) IC249.3(Q1)
MASK_5: IC228.9(C:I0) IC247.13(B:A2) IC249.4(Q2)
MASK_6: IC190.9(C:I0) IC247.15(B:A3) IC249.5(Q3)
MASK_7: IC242.9(C:I0)
MASK_ENABLE: IC116.5(A4) IC144.6(Q4) IC152.10(C:I1) IC190.10(C:I1) IC201.10(C:I1) IC203.10(C:I1) IC206.10(C:I1) IC228.10(C:I1) IC242.10(C:I1)
MASK_FLAGS_OUT: IC244.19(B:G) IC247.19(B:G)
MASK_FLAGS_WRT: IC248.1(M) IC248.2(N) IC249.1(M) IC249.2(N)
MDR_IN_BUS0: IC21.3(1D) IC180.3(1D)
MDR_IN_BUS1: IC21.4(2D) IC180.4(2D)
MDR_IN_BUS2: IC21.7(3D) IC180.7(3D)
MDR_IN_BUS3: IC21.8(4D) IC180.8(4D)
MDR_IN_BUS4: IC21.13(5D) IC180.13(5D)
MDR_IN_BUS5: IC21.14(6D) IC180.14(6D)
MDR_IN_BUS6: IC21.17(7D) IC180.17(7D)
MDR_IN_BUS7: IC21.18(8D) IC180.18(8D)
MDR_IN_SRC: IC22.1(!A!/B) IC23.1(!A!/B)
MDRH_DATA_OUT: IC178.1(A:G) IC179.1(A:G)
MDRH_WRT: IC180.1(G)
MDRH_X_OUT: IC176.1(A:G) IC181.1(A:G)
MDRH_Y_OUT: IC182.1(A:G) IC183.1(A:G)
MDRL_DATA_OUT: IC30.1(A:G) IC31.1(A:G)
MDRL_WRT: IC21.1(G)
MDRL_X_OUT: IC12.1(A:G) IC13.1(A:G)
MDRL_Y_OUT: IC10.1(A:G) IC11.1(A:G)
MEM_IO: IC69.5(B:Y3) RN4.14
N$1: IC1.2(1Q) IC117.2(A1)
N$2: IC1.5(2Q) IC117.3(A2)
N$3: IC1.6(3Q) IC117.4(A3)
N$4: IC1.9(4Q) IC117.5(A4)
N$5: IC1.12(5Q) IC117.6(A5)
N$6: IC1.15(6Q) IC117.7(A6)
N$7: IC102.8(A7) IC123.16(7Q)
N$8: IC1.19(8Q) IC117.9(A8)
N$9: IC139.1(M) IC139.2(N) IC147.6(B:O)
N$10: IC80.6(B:O) IC133.2(A:I1)
N$11: IC82.19(8Q) IC95.10(3B) IC104.9(A8) IC161.1(A:I0)
N$12: IC49.4(1Y) IC50.6(B1)
N$13: IC9.2(A1) IC100.2(1Q)
N$14: IC49.7(2Y) IC50.2(B2)
N$15: IC9.3(A2) IC100.5(2Q)
N$16: IC9.4(A3) IC100.6(3Q)
N$17: IC9.5(A4) IC100.9(4Q)
N$18: IC9.6(A5) IC100.12(5Q)
N$19: IC9.7(A6) IC100.15(6Q)
N$20: IC9.8(A7) IC100.16(7Q)
N$21: IC9.9(A8) IC100.19(8Q)
N$22: IC56.3(1C3) IC57.2(A:O)
N$23: IC65.1(A:O) IC138.1(A:I0)
N$24: IC143.3(A:O) IC170.5(B:I1)
N$25: IC2.2(A1) IC101.2(1Q)
N$26: IC2.3(A2) IC101.5(2Q)
N$27: IC2.4(A3) IC101.6(3Q)
N$28: IC2.5(A4) IC101.9(4Q)
N$29: IC2.6(A5) IC101.12(5Q)
N$30: IC2.7(A6) IC101.15(6Q)
N$31: IC2.8(A7) IC101.16(7Q)
N$32: IC2.9(A8) IC101.19(8Q)
N$33: IC56.4(1C2) IC57.1(A:I) IC167.4(1Y)
N$34: IC131.1(A:O) IC141.2(A:I1)
N$35: IC49.9(3Y) IC50.15(B3)
N$36: IC49.12(4Y) IC50.11(B4)
N$37: IC51.6(B1) IC55.4(1Y)
N$38: IC51.2(B2) IC55.7(2Y)
N$39: IC51.15(B3) IC55.9(3Y)
N$40: IC51.11(B4) IC55.12(4Y)
N$41: IC227.3(D1) IC241.7(1Y)
N$42: IC179.2(A:A1) IC180.2(1Q) IC181.2(A:A1) IC182.2(A:A1)
N$43: IC179.4(A:A2) IC180.5(2Q) IC181.4(A:A2) IC182.4(A:A2)
N$44: IC179.6(A:A3) IC180.6(3Q) IC181.6(A:A3) IC182.6(A:A3)
N$45: IC179.8(A:A4) IC180.9(4Q) IC181.8(A:A4) IC182.8(A:A4)
N$46: IC176.2(A:A1) IC178.2(A:A1) IC180.12(5Q) IC183.2(A:A1)
N$47: IC176.4(A:A2) IC178.4(A:A2) IC180.15(6Q) IC183.4(A:A2)
N$48: IC176.6(A:A3) IC178.6(A:A3) IC180.16(7Q) IC183.6(A:A3)
N$49: IC116.7(A6) IC128.4(Q2)
N$50: IC66.2(A:I0) IC130.6(B:O) IC143.2(A:I1)
N$51: IC176.8(A:A4) IC178.8(A:A4) IC180.19(8Q) IC183.8(A:A4)
N$52: IC27.15(B:A3) IC28.4(A3) IC189.6(3Q)
N$53: IC27.17(B:A4) IC28.5(A4) IC189.9(4Q)
N$54: IC26.11(B:A1) IC28.6(A5) IC189.12(5Q)
N$55: IC26.13(B:A2) IC28.7(A6) IC189.15(6Q)
N$56: IC26.15(B:A3) IC28.8(A7) IC189.16(7Q)
N$57: IC26.17(B:A4) IC28.9(A8) IC189.19(8Q)
N$58: IC7.2(1Q) IC25.11(B:A1) IC29.2(A1)
N$59: IC7.5(2Q) IC25.13(B:A2) IC29.3(A2)
N$60: IC7.6(3Q) IC25.15(B:A3) IC29.4(A3)
N$61: IC7.9(4Q) IC25.17(B:A4) IC29.5(A4)
N$62: IC7.12(5Q) IC24.11(B:A1) IC29.6(A5)
N$63: IC7.15(6Q) IC24.13(B:A2) IC29.7(A6)
N$64: IC7.16(7Q) IC24.15(B:A3) IC29.8(A7)
N$65: IC52.6(B1) IC63.4(1Y)
N$66: IC122.8(A7) IC227.19(Q8)
N$67: IC5.2(1Q) IC109.11(B:A1)
N$68: IC5.5(2Q) IC109.13(B:A2)
N$69: IC5.6(3Q) IC109.15(B:A3)
N$70: IC5.9(4Q) IC109.17(B:A4)
N$71: IC5.12(5Q) IC110.11(B:A1)
N$72: IC5.15(6Q) IC110.13(B:A2)
N$73: IC7.19(8Q) IC24.17(B:A4) IC29.9(A8)
N$74: IC52.2(B2) IC63.7(2Y)
N$75: IC52.15(B3) IC63.9(3Y)
N$76: IC44.3(A:CLK) IC139.7(CLK) SW3.C
N$77: IC75.3(D1) U$1.11(I/O0)
N$78: IC39.1(A:I0) IC43.4(B:O) IC45.1(A:I0)
N$79: IC32.3(D1) IC186.5(Y)
N$80: IC83.4(B:O) IC85.13(A:I2)
N$81: IC82.2(1Q) IC94.13(4B) IC104.2(A1)
N$82: IC66.1(A:O) IC170.4(B:I0)
N$83: IC10.2(A:A1) IC13.2(A:A1) IC21.2(1Q) IC30.2(A:A1)
N$84: IC133.1(A:I0) IC170.6(B:O)
N$85: IC66.3(A:I1) IC138.12(A:O)
N$86: IC59.1(A:I) IC209.6(B:O)
N$87: IC145.2(A1) IC184.2(1Q)
N$88: IC227.4(D2) IC243.7(1Y)
N$89: IC141.12(A:O) IC143.1(A:I0)
N$90: IC227.7(D3) IC255.7(1Y)
N$91: IC46.5(B:I1) IC47.3(A:O)
N$92: IC227.8(D4) IC256.7(1Y)
N$93: IC208.7(1Y) IC227.13(D5)
N$94: IC46.4(B:I0) IC119.4(B:O)
N$95: IC46.6(B:O) IC124.2(A:I1)
N$96: IC124.3(A:O) IC126.3(1D)
N$97: IC32.4(D2) IC160.5(Y)
N$98: IC257.4(1Y) RN5.16
N$99: IC257.7(2Y) RN5.15
N$100: IC257.9(3Y) RN5.14
N$101: IC257.12(4Y) RN5.13
N$102: IC258.4(1Y) RN5.12
N$103: IC258.7(2Y) RN5.11
N$104: IC258.9(3Y) RN5.10
N$105: IC258.12(4Y) RN5.9
N$106: IC99.19(8Q) IC114.9(A8)
N$107: IC14.16(CN+4) IC15.7(CN)
N$108: IC95.13(4B) IC161.3(A:O)
N$109: IC145.3(A2) IC184.5(2Q)
N$110: IC1.16(7Q) IC117.8(A7)
N$111: IC145.4(A3) IC184.6(3Q)
N$112: IC145.5(A4) IC184.9(4Q)
N$113: IC32.7(D3) IC159.5(Y)
N$114: IC86.2(1Q) IC89.2(A:A1)
N$115: IC86.5(2Q) IC89.4(A:A2)
N$116: IC86.6(3Q) IC89.6(A:A3)
N$117: IC86.9(4Q) IC89.8(A:A4)
N$118: IC86.12(5Q) IC90.2(A:A1)
N$119: IC86.15(6Q) IC90.4(A:A2)
N$120: IC86.16(7Q) IC90.6(A:A3)
N$121: IC86.19(8Q) IC90.8(A:A4)
N$122: IC88.2(1Q) IC91.2(A:A1)
N$123: IC88.5(2Q) IC91.4(A:A2)
N$124: IC88.6(3Q) IC91.6(A:A3)
N$125: IC88.9(4Q) IC91.8(A:A4)
N$126: IC88.12(5Q) IC92.2(A:A1)
N$127: IC88.15(6Q) IC92.4(A:A2)
N$128: IC88.16(7Q) IC92.6(A:A3)
N$129: IC88.19(8Q) IC92.8(A:A4)
N$130: IC42.2(A:I1) IC67.6(B:O)
N$131: IC93.3(1D) IC96.4(1Y)
N$132: IC10.4(A:A2) IC13.4(A:A2) IC21.5(2Q) IC30.4(A:A2)
N$133: IC45.3(A:O) IC67.5(B:I1)
N$134: IC10.6(A:A3) IC13.6(A:A3) IC21.6(3Q) IC30.6(A:A3)
N$135: IC145.6(A5) IC184.12(5Q)
N$136: IC145.7(A6) IC184.15(6Q)
N$137: IC10.8(A:A4) IC13.8(A:A4) IC21.9(4Q) IC30.8(A:A4)
N$138: IC11.2(A:A1) IC12.2(A:A1) IC21.12(5Q) IC31.2(A:A1)
N$139: IC145.8(A7) IC184.16(7Q)
N$140: IC11.4(A:A2) IC12.4(A:A2) IC21.15(6Q) IC31.4(A:A2)
N$141: IC11.6(A:A3) IC12.6(A:A3) IC21.16(7Q) IC31.6(A:A3)
N$142: IC145.9(A8) IC184.19(8Q)
N$143: IC5.16(7Q) IC110.15(B:A3)
N$144: IC52.11(B4) IC63.12(4Y)
N$145: IC53.6(B1) IC68.4(1Y)
N$146: IC5.19(8Q) IC110.17(B:A4)
N$147: IC53.2(B2) IC68.7(2Y)
N$148: IC93.4(2D) IC96.7(2Y)
N$149: IC93.7(3D) IC96.9(3Y)
N$150: IC55.13(4B) IC63.3(1B) IC63.6(2B) IC63.10(3B) IC63.13(4B) IC68.3(1B) IC68.6(2B)
N$151: IC4.2(1Q) IC111.11(B:A1)
N$152: IC49.1(!A!/B) IC55.1(!A!/B) IC63.1(!A!/B) IC68.1(!A!/B) IC85.12(A:O)
N$153: IC32.8(D4) IC142.5(Y)
N$154: IC84.4(B:O) IC85.2(A:I1)
N$155: IC116.8(A7) IC128.5(Q3)
N$156: IC93.8(4D) IC96.12(4Y)
N$157: IC93.13(5D) IC94.4(1Y)
N$158: IC93.14(6D) IC94.7(2Y)
N$159: IC93.17(7D) IC94.9(3Y)
N$160: IC93.18(8D) IC94.12(4Y)
N$161: IC82.3(1D) IC97.4(1Y)
N$162: IC82.4(2D) IC97.7(2Y)
N$163: IC82.7(3D) IC97.9(3Y)
N$164: IC11.8(A:A4) IC12.8(A:A4) IC21.19(8Q) IC31.8(A:A4)
N$165: IC82.8(4D) IC97.12(4Y)
N$166: IC82.13(5D) IC95.4(1Y)
N$167: SW3.2
N$168: IC82.14(6D) IC95.7(2Y)
N$169: IC10.18(A:Y1)
N$170: IC10.16(A:Y2)
N$171: IC10.14(A:Y3)
N$172: IC10.12(A:Y4)
N$173: IC82.17(7D) IC95.9(3Y)
N$174: IC32.13(D5) IC129.5(Y)
N$175: IC32.14(D6) IC73.5(Y)
N$176: IC14.7(CN) IC56.7(1Y)
N$177: IC13.18(A:Y1)
N$178: IC13.16(A:Y2)
N$179: IC13.14(A:Y3)
N$180: IC13.12(A:Y4)
N$181: IC12.18(A:Y1)
N$182: IC12.16(A:Y2)
N$183: IC12.14(A:Y3)
N$184: IC12.12(A:Y4)
N$185: IC32.17(D7) IC34.5(Y)
N$186: IC32.18(D8) IC35.5(Y)
N$187: IC33.3(D1) IC36.5(Y)
N$188: IC33.4(D2) IC37.5(Y)
N$189: IC33.7(D3) IC38.5(Y)
N$190: IC33.8(D4) IC40.5(Y)
N$191: IC22.7(2Y)
N$192: IC22.9(3Y)
N$193: IC22.12(4Y)
N$194: IC23.4(1Y)
N$195: IC23.7(2Y)
N$196: IC23.9(3Y)
N$197: IC23.12(4Y)
N$198: IC22.3(1B)
N$199: IC22.6(2B)
N$200: IC30.18(A:Y1)
N$201: IC30.16(A:Y2)
N$202: IC82.18(8D) IC95.12(4Y)
N$203: IC30.14(A:Y3)
N$204: IC30.12(A:Y4)
N$205: IC82.16(7Q) IC95.6(2B) IC104.8(A7)
N$206: IC31.18(A:Y1)
N$207: IC31.16(A:Y2)
N$208: IC31.14(A:Y3)
N$209: IC31.12(A:Y4)
N$210: IC22.4(1Y)
N$211: IC22.10(3B)
N$212: IC22.13(4B)
N$213: IC23.3(1B)
N$214: IC23.6(2B)
N$215: IC23.10(3B)
N$216: IC23.13(4B)
N$217: IC116.9(A8) IC128.6(Q4)
N$218: IC33.13(D5) IC41.5(Y)
N$219: IC33.14(D6) IC71.5(Y)
N$220: IC148.3(A:O) IC162.3(D1)
N$221: IC102.6(A5) IC123.12(5Q)
N$222: IC195.2(A:I1) IC222.15(Y0)
N$223: IC8.1(A:CLR) IC195.3(A:O)
N$224: IC8.5(A:Q) IC148.2(A:I1)
N$225: IC20.5(Y) IC33.17(D7)
N$226: IC196.4(B:O) IC226.4
N$227: IC39.3(A:O)
N$228: IC33.18(D8) IC172.5(Y)
N$229: IC102.7(A6) IC123.15(6Q)
N$230: IC205.2(1Q) IC210.2(A1)
N$231: IC120.3(A:O) IC241.4(1C2)
N$232: IC82.15(6Q) IC95.3(1B) IC104.7(A6)
N$233: IC82.12(5Q) IC97.13(4B) IC104.6(A5)
N$234: IC205.5(2Q) IC210.3(A2)
N$235: IC102.9(A8) IC123.19(8Q)
N$236: IC102.2(A1) IC123.2(1Q)
N$237: IC102.3(A2) IC123.5(2Q)
N$238: IC102.4(A3) IC123.6(3Q)
N$239: IC205.6(3Q) IC210.4(A3)
N$240: IC205.9(4Q) IC210.5(A4)
N$241: IC205.12(5Q) IC210.6(A5)
N$242: IC205.15(6Q) IC210.7(A6)
N$243: IC205.16(7Q) IC210.8(A7)
N$244: IC205.19(8Q) IC210.9(A8)
N$245: IC140.2(A1) IC173.2(1Q)
N$246: IC140.3(A2) IC173.5(2Q)
N$247: IC140.4(A3) IC173.6(3Q)
N$248: IC140.5(A4) IC173.9(4Q)
N$249: IC102.5(A4) IC123.9(4Q)
N$250: IC140.6(A5) IC173.12(5Q)
N$251: U$2.10(A0)
N$252: U$2.9(A1)
N$253: U$2.8(A2)
N$254: U$2.7(A3)
N$255: U$2.6(A4)
N$256: U$2.5(A5)
N$257: U$2.4(A6)
N$258: U$2.3(A7)
N$259: U$2.25(A8)
N$260: U$2.24(A9)
N$261: U$2.21(A10)
N$262: U$2.23(A11)
N$263: U$2.2(A12)
N$264: U$2.26(A13)
N$265: U$3.10(A0)
N$266: U$3.9(A1)
N$267: U$3.8(A2)
N$268: U$3.7(A3)
N$269: U$3.6(A4)
N$270: U$3.5(A5)
N$271: U$3.4(A6)
N$272: U$3.3(A7)
N$273: U$3.25(A8)
N$274: U$3.24(A9)
N$275: U$3.21(A10)
N$276: U$3.23(A11)
N$277: U$3.2(A12)
N$278: U$3.26(A13)
N$279: U$4.10(A0)
N$280: U$4.9(A1)
N$281: U$4.8(A2)
N$282: U$4.7(A3)
N$283: U$4.6(A4)
N$284: U$4.5(A5)
N$285: U$4.4(A6)
N$286: U$4.3(A7)
N$287: U$4.25(A8)
N$288: U$4.24(A9)
N$289: U$4.21(A10)
N$290: U$4.23(A11)
N$291: U$4.2(A12)
N$292: U$4.26(A13)
N$293: U$5.10(A0)
N$294: U$5.9(A1)
N$295: U$5.8(A2)
N$296: U$5.7(A3)
N$297: U$5.6(A4)
N$298: U$5.5(A5)
N$299: U$5.4(A6)
N$300: U$5.3(A7)
N$301: U$5.25(A8)
N$302: U$5.24(A9)
N$303: U$5.21(A10)
N$304: U$5.23(A11)
N$305: U$5.2(A12)
N$306: U$5.26(A13)
N$307: IC140.7(A6) IC173.15(6Q)
N$308: IC140.8(A7) IC173.16(7Q)
N$309: IC140.9(A8) IC173.19(8Q)
N$310: IC166.2(1Q) IC171.2(A1)
N$311: IC166.5(2Q) IC171.3(A2)
N$312: IC82.9(4Q) IC97.10(3B) IC104.5(A4)
N$313: IC82.6(3Q) IC97.6(2B) IC104.4(A3)
N$314: IC82.5(2Q) IC97.3(1B) IC104.3(A2)
N$315: IC166.6(3Q) IC171.4(A3)
N$316: IC93.19(8Q) IC94.10(3B) IC103.9(A8)
N$317: IC93.16(7Q) IC94.6(2B) IC103.8(A7)
N$318: IC93.15(6Q) IC94.3(1B) IC103.7(A6)
N$319: IC93.12(5Q) IC96.13(4B) IC103.6(A5)
N$320: IC154.7(A6) IC226.9(A0)
N$321: IC93.9(4Q) IC96.10(3B) IC103.5(A4)
N$322: IC175.6(B:O) IC177.4(B:I0)
N$323: IC93.6(3Q) IC96.6(2B) IC103.4(A3)
N$324: IC177.6(B:O) IC192.4(B:I0)
N$325: IC3.2(A1) IC153.2(1Q)
N$326: IC3.3(A2) IC153.5(2Q)
N$327: IC3.4(A3) IC153.6(3Q)
N$328: IC3.5(A4) IC153.9(4Q)
N$329: IC3.6(A5) IC153.12(5Q)
N$330: IC3.7(A6) IC153.15(6Q)
N$331: IC3.8(A7) IC153.16(7Q)
N$332: IC3.9(A8) IC153.19(8Q)
N$333: IC50.5(A1)
N$334: IC50.3(A2)
N$335: IC50.14(A3)
N$336: IC50.12(A4)
N$337: IC52.5(A1)
N$338: IC51.5(A1)
N$339: IC51.3(A2)
N$340: IC51.14(A3)
N$341: IC51.12(A4)
N$342: IC146.2(A1) IC185.2(1Q)
N$343: IC93.5(2Q) IC96.3(1B) IC103.3(A2)
N$344: IC166.9(4Q) IC171.5(A4)
N$345: IC166.12(5Q) IC171.6(A5)
N$346: IC158.1(A:I0) IC190.8(C:O)
N$347: IC121.3(1B) IC127.3(A:O)
N$348: IC125.2(A1) IC162.2(Q1) IC196.3(B:I)
N$349: IC149.3(B:I) IC226.14(GS)
N$350: IC52.3(A2)
N$351: IC52.14(A3)
N$352: IC52.12(A4)
N$353: IC53.5(A1)
N$354: IC53.3(A2)
N$355: IC158.12(A:O) IC226.11
N$356: IC149.4(B:O) IC202.2(A:I1)
N$357: IC50.9(C4) IC51.7(C0)
N$358: IC51.9(C4) IC52.7(C0)
N$359: IC52.9(C4) IC53.7(C0)
N$360: IC76.5(Q2)
N$361: IC202.1(A:I0) IC226.15(EO)
N$362: IC192.6(B:O) IC193.4(B:I0)
N$363: IC166.15(6Q) IC171.7(A6)
N$364: IC76.6(Q3)
N$365: IC64.12(A:O) IC226.3
N$366: IC64.13(A:I2) IC125.3(A2) IC162.5(Q2)
N$367: IC75.4(D2) U$1.12(I/O1)
N$368: IC132.1(A:I0) IC201.8(C:O)
N$369: IC75.7(D3) U$1.13(I/O2)
N$370: IC166.16(7Q) IC171.8(A7)
N$371: IC166.19(8Q) IC171.9(A8)
N$372: IC168.1(A:CLR) IC220.3(A:O)
N$373: IC146.3(A2) IC185.5(2Q)
N$374: IC174.1(A:CLR) IC223.3(A:O)
N$375: IC75.8(D4) U$1.15(I/O3)
N$376: IC75.13(D5) U$1.16(I/O4)
N$377: IC75.14(D6) U$1.17(I/O5)
N$378: IC60.3(D1) U$10.11(I/O0)
N$379: IC60.4(D2) U$10.12(I/O1)
N$380: IC60.7(D3) U$10.13(I/O2)
N$381: IC60.8(D4) U$10.15(I/O3)
N$382: IC60.13(D5) U$10.16(I/O4)
N$383: IC60.14(D6) U$10.17(I/O5)
N$384: IC60.17(D7) U$10.18(I/O6)
N$385: IC60.18(D8) U$10.19(I/O7)
N$386: IC61.3(D1) U$11.11(I/O0)
N$387: IC61.4(D2) U$11.12(I/O1)
N$388: IC188.1(A:CLR) IC224.3(A:O)
N$389: IC162.18(D8) IC187.5(A:Q)
N$390: IC162.4(D2) IC163.5(A:Q)
N$391: IC76.9(Q4)
N$392: IC162.7(D3) IC164.5(A:Q)
N$393: IC162.8(D4) IC168.5(A:Q)
N$394: IC162.13(D5) IC174.5(A:Q)
N$395: IC162.14(D6) IC188.5(A:Q)
N$396: IC162.17(D7) IC221.5(A:Q)
N$397: IC207.1(A:I0) IC222.7(Y7)
N$398: IC218.2(A:I1) IC222.14(Y1)
N$399: IC219.2(A:I1) IC222.13(Y2)
N$400: IC76.12(Q5)
N$401: IC76.15(Q6)
N$402: IC76.16(Q7)
N$403: IC222.11(Y4) IC223.1(A:I0)
N$404: IC4.5(2Q) IC111.13(B:A2)
N$405: IC222.9(Y6) IC225.1(A:I0)
N$406: IC187.1(A:CLR) IC207.3(A:O)
N$408: IC163.1(A:CLR) IC218.3(A:O)
N$409: IC164.1(A:CLR) IC219.3(A:O)
N$410: IC221.1(A:CLR) IC225.3(A:O)
N$411: IC125.4(A3) IC132.13(A:I2) IC162.6(Q3)
N$412: IC125.5(A4) IC150.13(A:I2) IC162.9(Q4)
N$413: IC132.12(A:O) IC226.2
N$414: IC125.6(A5) IC151.13(A:I2) IC162.12(Q5)
N$415: IC150.1(A:I0) IC203.8(C:O)
N$416: IC150.12(A:O) IC226.1
N$417: IC151.1(A:I0) IC206.8(C:O)
N$418: IC151.12(A:O) IC226.13
N$419: IC157.1(A:I0) IC228.8(C:O)
N$420: IC157.12(A:O) IC226.12
N$421: IC191.1(A:I0) IC242.8(C:O)
N$422: IC146.4(A3) IC185.6(3Q)
N$423: IC146.5(A4) IC185.9(4Q)
N$424: IC146.6(A5) IC185.12(5Q)
N$425: IC146.7(A6) IC185.15(6Q)
N$426: IC146.8(A7) IC185.16(7Q)
N$427: IC146.9(A8) IC185.19(8Q)
N$428: IC216.2(1Q) IC245.2(A1)
N$429: IC216.5(2Q) IC245.3(A2)
N$430: IC216.6(3Q) IC245.4(A3)
N$431: IC216.9(4Q) IC245.5(A4)
N$432: IC216.12(5Q) IC245.6(A5)
N$433: IC216.15(6Q) IC245.7(A6)
N$434: IC216.16(7Q) IC245.8(A7)
N$435: IC216.19(8Q) IC245.9(A8)
N$436: IC191.12(A:O) IC226.10
N$437: IC125.7(A6) IC157.13(A:I2) IC162.15(Q6)
N$438: IC125.8(A7) IC158.13(A:I2) IC162.16(Q7)
N$439: IC125.9(A8) IC162.19(Q8) IC191.13(A:I2)
N$440: IC76.19(Q8)
N$441: IC165.2(1Q) IC215.2(A1)
N$442: IC76.3(D1) U$2.11(I/O0)
N$443: IC76.4(D2) U$2.12(I/O1)
N$444: IC247.17(B:A4) IC249.6(Q4)
N$445: IC193.6(B:O) IC194.4(B:I0)
N$446: IC197.5(A:O) IC198.1(A:I)
N$447: IC77.5(Q2)
N$448: IC61.7(D3) U$11.13(I/O2)
N$449: IC75.17(D7) U$1.18(I/O6)
N$450: IC75.18(D8) U$1.19(I/O7)
N$451: IC76.7(D3) U$2.13(I/O2)
N$452: IC76.8(D4) U$2.15(I/O3)
N$453: IC76.13(D5) U$2.16(I/O4)
N$454: IC76.14(D6) U$2.17(I/O5)
N$455: IC76.17(D7) U$2.18(I/O6)
N$456: IC76.18(D8) U$2.19(I/O7)
N$457: IC77.3(D1) U$3.11(I/O0)
N$458: IC77.4(D2) U$3.12(I/O1)
N$459: IC77.7(D3) U$3.13(I/O2)
N$460: IC77.8(D4) U$3.15(I/O3)
N$461: IC77.13(D5) U$3.16(I/O4)
N$462: IC77.14(D6) U$3.17(I/O5)
N$463: IC77.17(D7) U$3.18(I/O6)
N$464: IC77.18(D8) U$3.19(I/O7)
N$465: IC78.3(D1) U$4.11(I/O0)
N$466: IC78.4(D2) U$4.12(I/O1)
N$467: IC78.7(D3) U$4.13(I/O2)
N$468: IC78.8(D4) U$4.15(I/O3)
N$469: IC78.13(D5) U$4.16(I/O4)
N$470: IC78.14(D6) U$4.17(I/O5)
N$471: IC78.17(D7) U$4.18(I/O6)
N$472: IC78.18(D8) U$4.19(I/O7)
N$473: IC79.3(D1) U$5.11(I/O0)
N$474: IC79.4(D2) U$5.12(I/O1)
N$475: IC79.7(D3) U$5.13(I/O2)
N$476: IC79.8(D4) U$5.15(I/O3)
N$477: IC79.13(D5) U$5.16(I/O4)
N$478: IC79.14(D6) U$5.17(I/O5)
N$479: IC79.17(D7) U$5.18(I/O6)
N$480: IC79.18(D8) U$5.19(I/O7)
N$481: IC198.2(A:O) IC199.1(A:I0)
N$482: IC61.8(D4) U$11.15(I/O3)
N$483: IC61.13(D5) U$11.16(I/O4)
N$484: IC61.14(D6) U$11.17(I/O5)
N$485: IC61.17(D7) U$11.18(I/O6)
N$486: IC61.18(D8) U$11.19(I/O7)
N$487: IC62.3(D1) U$12.11(I/O0)
N$488: IC62.4(D2) U$12.12(I/O1)
N$489: IC62.7(D3) U$12.13(I/O2)
N$490: IC62.8(D4) U$12.15(I/O3)
N$491: IC62.13(D5) U$12.16(I/O4)
N$492: IC62.14(D6) U$12.17(I/O5)
N$493: IC62.17(D7) U$12.18(I/O6)
N$494: IC62.18(D8) U$12.19(I/O7)
N$495: IC194.6(B:O) IC200.4(B:I0)
N$496: IC200.6(B:O) IC209.4(B:I0)
N$497: IC165.5(2Q) IC215.3(A2)
N$498: IC165.6(3Q) IC215.4(A3)
N$499: IC165.9(4Q) IC215.5(A4)
N$500: IC165.12(5Q) IC215.6(A5)
N$501: IC165.15(6Q) IC215.7(A6)
N$502: IC165.16(7Q) IC215.8(A7)
N$503: IC134.18(D8) U$6.19(I/O7)
N$504: IC134.17(D7) U$6.18(I/O6)
N$505: IC134.14(D6) U$6.17(I/O5)
N$506: IC134.13(D5) U$6.16(I/O4)
N$507: IC134.8(D4) U$6.15(I/O3)
N$508: IC134.7(D3) U$6.13(I/O2)
N$509: IC134.4(D2) U$6.12(I/O1)
N$510: IC134.3(D1) U$6.11(I/O0)
N$511: IC135.3(D1) U$7.11(I/O0)
N$512: IC135.4(D2) U$7.12(I/O1)
N$513: IC135.7(D3) U$7.13(I/O2)
N$514: IC135.8(D4) U$7.15(I/O3)
N$515: IC135.13(D5) U$7.16(I/O4)
N$516: IC135.14(D6) U$7.17(I/O5)
N$517: IC135.17(D7) U$7.18(I/O6)
N$518: IC135.18(D8) U$7.19(I/O7)
N$519: IC136.3(D1) U$8.11(I/O0)
N$520: IC136.4(D2) U$8.12(I/O1)
N$521: IC136.7(D3) U$8.13(I/O2)
N$522: IC136.8(D4) U$8.15(I/O3)
N$523: IC136.13(D5) U$8.16(I/O4)
N$524: IC136.14(D6) U$8.17(I/O5)
N$525: IC136.17(D7) U$8.18(I/O6)
N$526: IC136.18(D8) U$8.19(I/O7)
N$527: IC137.3(D1) U$9.11(I/O0)
N$528: IC87.3(A:S2) R1.1 S1.1(O)
N$529: IC87.1(A:R) R2.1 S1.3(S)
N$531: IC87.4(A:Q) SW3.1
N$532: SW3.4
N$533: IC137.4(D2) U$9.12(I/O1)
N$534: IC137.7(D3) U$9.13(I/O2)
N$535: IC137.8(D4) U$9.15(I/O3)
N$536: IC137.13(D5) U$9.16(I/O4)
N$537: IC137.14(D6) U$9.17(I/O5)
N$538: IC137.17(D7) U$9.18(I/O6)
N$539: IC137.18(D8) U$9.19(I/O7)
N$541: IC64.1(A:I0) IC152.8(C:O)
N$542: IC165.19(8Q) IC215.9(A8)
N$543: IC246.2(1Q) IC259.2(A1)
N$544: IC246.5(2Q) IC259.3(A2)
N$545: IC246.6(3Q) IC259.4(A3)
N$546: IC246.9(4Q) IC259.5(A4)
N$547: IC246.12(5Q) IC259.6(A5)
N$548: IC57.3(B:I) IC139.3(Q1)
N$549: IC246.15(6Q) IC259.7(A6)
N$550: IC246.16(7Q) IC259.8(A7)
N$551: IC246.19(8Q) IC259.9(A8)
N$552: IC217.2(1Q) IC260.2(A1)
N$553: IC217.5(2Q) IC260.3(A2)
N$554: IC217.6(3Q) IC260.4(A3)
N$555: IC217.9(4Q) IC260.5(A4)
N$556: IC217.12(5Q) IC260.6(A5)
N$557: IC217.15(6Q) IC260.7(A6)
N$558: IC217.16(7Q) IC260.8(A7)
N$559: IC217.19(8Q) IC260.9(A8)
N$560: IC262.2(1Q) IC263.2(A1)
N$561: IC262.5(2Q) IC263.3(A2)
N$562: IC262.6(3Q) IC263.4(A3)
N$563: IC262.9(4Q) IC263.5(A4)
N$564: IC77.6(Q3)
N$565: IC262.12(5Q) IC263.6(A5)
N$566: IC262.15(6Q) IC263.7(A6)
N$567: IC70.13(D6) IC81.6(B:O)
N$568: IC77.9(Q4)
N$569: IC18.6(B:O) IC70.12(D7)
N$570: IC262.16(7Q) IC263.8(A7)
N$571: IC77.12(Q5)
N$572: IC262.19(8Q) IC263.9(A8)
N$573: IC261.2(1Q) IC264.2(A1)
N$574: IC16.2(1Q) IC211.2(A:A1)
N$575: IC16.5(2Q) IC211.4(A:A2)
N$576: IC16.6(3Q) IC211.6(A:A3)
N$577: IC4.6(3Q) IC111.15(B:A3)
N$578: IC4.9(4Q) IC111.17(B:A4)
N$579: IC4.12(5Q) IC112.11(B:A1)
N$580: IC4.15(6Q) IC112.13(B:A2)
N$581: IC4.16(7Q) IC112.15(B:A3)
N$582: IC4.19(8Q) IC112.17(B:A4)
N$583: IC98.2(1Q) IC113.2(A1)
N$584: IC98.5(2Q) IC113.3(A2)
N$585: IC98.6(3Q) IC113.4(A3)
N$586: IC98.9(4Q) IC113.5(A4)
N$587: IC98.12(5Q) IC113.6(A5)
N$588: IC98.15(6Q) IC113.7(A6)
N$589: IC98.16(7Q) IC113.8(A7)
N$590: IC98.19(8Q) IC113.9(A8)
N$591: IC99.2(1Q) IC114.2(A1)
N$592: IC99.5(2Q) IC114.3(A2)
N$593: IC99.6(3Q) IC114.4(A3)
N$594: IC99.9(4Q) IC114.5(A4)
N$595: IC99.12(5Q) IC114.6(A5)
N$596: IC99.15(6Q) IC114.7(A6)
N$597: IC99.16(7Q) IC114.8(A7)
N$598: IC261.5(2Q) IC264.3(A2)
N$599: IC261.6(3Q) IC264.4(A3)
N$600: IC261.9(4Q) IC264.5(A4)
N$601: IC16.9(4Q) IC211.8(A:A4)
N$602: IC77.15(Q6)
N$603: IC16.12(5Q) IC212.2(A:A1)
N$604: IC16.15(6Q) IC212.4(A:A2)
N$605: IC77.16(Q7)
N$606: IC77.19(Q8)
N$607: IC261.12(5Q) IC264.6(A5)
N$608: IC261.15(6Q) IC264.7(A6)
N$609: IC261.16(7Q) IC264.8(A7)
N$610: IC261.19(8Q) IC264.9(A8)
N$655: IC16.16(7Q) IC212.6(A:A3)
N$656: IC16.19(8Q) IC212.8(A:A4)
N$657: IC17.2(1Q) IC213.2(A:A1)
N$658: IC17.5(2Q) IC213.4(A:A2)
N$659: IC17.6(3Q) IC213.6(A:A3)
N$660: IC17.9(4Q) IC213.8(A:A4)
N$661: IC17.12(5Q) IC214.2(A:A1)
N$662: IC17.15(6Q) IC214.4(A:A2)
N$663: IC17.16(7Q) IC214.6(A:A3)
N$664: IC17.19(8Q) IC214.8(A:A4)
N$685: IC220.1(A:I0) IC222.12(Y3)
N$687: IC222.10(Y5) IC224.1(A:I0)
N$688: IC229.2(A:A1) IC234.2(1Q)
N$689: IC229.4(A:A2) IC234.5(2Q)
N$690: IC229.6(A:A3) IC234.6(3Q)
N$691: IC230.2(A:A1) IC234.12(5Q)
N$692: IC230.4(A:A2) IC234.15(6Q)
N$693: IC230.6(A:A3) IC234.16(7Q)
N$694: IC230.8(A:A4) IC234.19(8Q)
N$695: IC231.2(A:A1) IC233.2(1Q)
N$696: IC231.4(A:A2) IC233.5(2Q)
N$697: IC231.6(A:A3) IC233.6(3Q)
N$698: IC231.8(A:A4) IC233.9(4Q)
N$699: IC232.2(A:A1) IC233.12(5Q)
N$700: IC232.4(A:A2) IC233.15(6Q)
N$701: IC232.6(A:A3) IC233.16(7Q)
N$702: IC232.8(A:A4) IC233.19(8Q)
N$703: IC230.1(A:G)
N$704: IC234.9(4Q)
N$705: IC235.2(A:A1) IC240.2(1Q)
N$706: IC235.4(A:A2) IC240.5(2Q)
N$707: IC235.6(A:A3) IC240.6(3Q)
N$708: IC236.2(A:A1) IC240.12(5Q)
N$709: IC236.4(A:A2) IC240.15(6Q)
N$710: IC236.6(A:A3) IC240.16(7Q)
N$711: IC236.8(A:A4) IC240.19(8Q)
N$712: IC237.2(A:A1) IC239.2(1Q)
N$713: IC237.4(A:A2) IC239.5(2Q)
N$714: IC237.6(A:A3) IC239.6(3Q)
N$715: IC237.8(A:A4) IC239.9(4Q)
N$716: IC238.2(A:A1) IC239.12(5Q)
N$717: IC238.4(A:A2) IC239.15(6Q)
N$718: IC238.6(A:A3) IC239.16(7Q)
N$719: IC238.8(A:A4) IC239.19(8Q)
N$720: IC236.1(A:G)
N$721: IC240.9(4Q)
NOT_CONDITION: IC74.4(B:I0)
NOT_RST: IC75.1(CLR) IC76.1(CLR) IC77.1(CLR) IC78.1(CLR) IC79.1(CLR) IC134.1(CLR) IC135.1(CLR) IC136.1(CLR) IC137.1(CLR)
OF: IC122.5(A4) IC156.10(2C0) IC227.9(Q4) IC256.6(1C0)
OF_FROM_ALU: IC126.8(4D) IC156.12(2C2) IC256.5(1C1)
OF_IN_SRC_0: IC256.14(A)
OF_IN_SRC_1: IC256.2(B)
PANEL_MEM_IO: RN4.3
PANEL_RD: RN4.1
PANEL_WR: RN4.2
PCH_0: IC6.2(1Q) IC107.11(B:A1)
PCH_1: IC6.5(2Q) IC107.13(B:A2)
PCH_2: IC6.6(3Q) IC107.15(B:A3)
PCH_3: IC6.9(4Q) IC107.17(B:A4)
PCH_4: IC6.12(5Q) IC108.11(B:A1)
PCH_5: IC6.15(6Q) IC108.13(B:A2)
PCH_6: IC6.16(7Q) IC108.15(B:A3)
PCH_7: IC6.19(8Q) IC108.17(B:A4)
PCH_OUT: IC107.19(B:G) IC108.19(B:G)
PCH_WRT: IC6.1(G)
PCL_0: IC48.2(1Q) IC105.11(B:A1)
PCL_1: IC48.5(2Q) IC105.13(B:A2)
PCL_2: IC48.6(3Q) IC105.15(B:A3)
PCL_3: IC48.9(4Q) IC105.17(B:A4)
PCL_4: IC48.12(5Q) IC106.11(B:A1)
PCL_5: IC48.15(6Q) IC106.13(B:A2)
PCL_6: IC48.16(7Q) IC106.15(B:A3)
PCL_7: IC48.19(8Q) IC106.17(B:A4)
PCL_OUT: IC105.19(B:G) IC106.19(B:G)
PCL_WRT: IC48.1(G)
PF: IC70.15(D4) IC122.9(A8) IC208.6(1C0) IC227.12(Q5)
PF_FROM_ALU: IC59.2(A:O) IC208.5(1C1)
PF_IN_SRC_0: IC208.14(A)
PF_IN_SRC_1: IC208.2(B)
PROG_MODE: IC250.5(B:I1)
RD: IC69.9(B:Y1) RN4.16
REQ_ENCOD_0: IC222.1(A)
REQ_ENCOD_1: IC154.6(A5) IC222.2(B) IC226.7(A1)
REQ_ENCOD_2: IC154.5(A4) IC222.3(C) IC226.6(A2)
RST: IC54.3(B:I) IC128.15(CLR) IC139.15(CLR) IC144.15(CLR) IC248.15(CLR) IC249.15(CLR) R3.1 S2.2(P)
SF: IC122.4(A3) IC156.6(1C0) IC227.6(Q3) IC255.6(1C0)
SF_FROM_ALU: IC126.7(3D) IC156.4(1C2)
SF_IN_SRC_0: IC255.14(A)
SF_IN_SRC_1: IC255.2(B)
SF_XOR_OF: IC70.14(D5) IC72.6(B:O) IC81.4(B:I0)
SHR_MACHINE_H_OUT: IC104.1(G1) IC104.19(G2)
SHR_MACHINE_H_WRT: IC82.1(G)
SHR_MACHINE_IN_SRC: IC94.1(!A!/B) IC95.1(!A!/B) IC96.1(!A!/B) IC97.1(!A!/B)
SHR_MACHINE_L_OUT: IC103.1(G1) IC103.19(G2)
SHR_MACHINE_L_WRT: IC93.1(G)
SHR_MACHINE_TYPE: IC161.2(A:I1)
SPH_OUT: IC111.19(B:G) IC112.19(B:G)
SPH_WRT: IC4.1(G)
SPL_OUT: IC109.19(B:G) IC110.19(B:G)
SPL_WRT: IC5.1(G)
SS_H_OUT: IC260.1(G1) IC260.19(G2)
SS_H_WRT: IC217.1(G)
SS_L_OUT: IC259.1(G1) IC259.19(G2)
SS_L_WRT: IC246.1(G)
STOP_CLK: IC44.2(A:D) IC44.5(A:Q) IC147.4(B:I0) R9.1 S4.2(P)
TDR0_H_WRT: IC239.1(G)
TDR0_H_X_OUT: IC237.1(A:G) IC238.1(A:G)
TDR0_L_WRT: IC240.1(G)
TDR0_L_X_OUT: IC235.8(A:A4)
TDR0H_WRT: IC17.1(G)
TDR0H_Y_OUT: IC213.1(A:G) IC214.1(A:G)
TDR0L_OUT3: IC229.1(A:G)
TDR0L_OUT4: IC235.1(A:G)
TDR0L_WRT: IC16.1(G)
TDR0L_Y_OUT: IC211.1(A:G) IC212.1(A:G)
TDR1_H_WRT: IC233.1(G)
TDR1_H_X_OUT: IC231.1(A:G) IC232.1(A:G)
TDR1_L_WRT: IC234.1(G)
TDR1_L_X_OUT: IC229.8(A:A4)
TDR1H_WRT: IC88.1(G)
TDR1H_Y_OUT: IC91.1(A:G) IC92.1(A:G)
TDR1L_WRT: IC86.1(G)
TDR1L_Y_OUT: IC89.1(A:G) IC90.1(A:G)
TRAP: IC45.2(A:I1)
TRAP_REQ: IC8.3(A:CLK) IC148.1(A:I0) R5.2
TYP_0: IC43.3(B:I) IC67.4(B:I0) IC85.1(A:I0)
TYP_1: IC39.2(A:I1) IC42.1(A:I0) IC84.3(B:I)
U_AD0: IC32.2(Q1) U$6.10(A0) U$7.10(A0) U$8.10(A0) U$9.10(A0)
U_AD1: IC32.5(Q2) U$6.9(A1) U$7.9(A1) U$8.9(A1) U$9.9(A1)
U_AD2: IC32.6(Q3) U$6.8(A2) U$7.8(A2) U$8.8(A2) U$9.8(A2)
U_AD3: IC32.9(Q4) U$6.7(A3) U$7.7(A3) U$8.7(A3) U$9.7(A3)
U_AD4: IC32.12(Q5) U$6.6(A4) U$7.6(A4) U$8.6(A4) U$9.6(A4)
U_AD5: IC32.15(Q6) U$6.5(A5) U$7.5(A5) U$8.5(A5) U$9.5(A5)
U_AD6: IC32.16(Q7) U$6.4(A6) U$7.4(A6) U$8.4(A6) U$9.4(A6)
U_AD7: IC32.19(Q8) U$6.3(A7) U$7.3(A7) U$8.3(A7) U$9.3(A7)
U_AD8: IC33.2(Q1) U$6.25(A8) U$7.25(A8) U$8.25(A8) U$9.25(A8)
U_AD9: IC33.5(Q2) U$6.24(A9) U$7.24(A9) U$8.24(A9) U$9.24(A9)
U_AD10: IC33.6(Q3) U$6.21(A10) U$7.21(A10) U$8.21(A10) U$9.21(A10)
U_AD11: IC33.9(Q4) U$6.23(A11) U$7.23(A11) U$8.23(A11) U$9.23(A11)
U_AD12: IC33.12(Q5) U$6.2(A12) U$7.2(A12) U$8.2(A12) U$9.2(A12)
U_AD13: IC33.15(Q6) U$6.26(A13) U$7.26(A13) U$8.26(A13) U$9.26(A13)
U_AD14: IC33.16(Q7)
U_AD15: IC33.19(Q8)
U_AD_BUFF0: U$1.10(A0)
U_AD_BUFF1: U$1.9(A1)
U_AD_BUFF2: U$1.8(A2)
U_AD_BUFF3: U$1.7(A3)
U_AD_BUFF4: U$1.6(A4)
U_AD_BUFF5: U$1.5(A5)
U_AD_BUFF6: U$1.4(A6)
U_AD_BUFF7: U$1.3(A7)
U_AD_BUFF8: U$1.25(A8)
U_AD_BUFF9: U$1.24(A9)
U_AD_BUFF10: U$1.21(A10)
U_AD_BUFF11: U$1.23(A11)
U_AD_BUFF12: U$1.2(A12)
U_AD_BUFF13: U$1.26(A13)
U_ADDER_0: IC50.4(S1) IC186.4(D0)
U_ADDER_1: IC160.4(D0)
U_ADDER_2: IC159.4(D0)
U_ADDER_3: IC142.4(D0)
U_ADDER_4: IC129.4(D0)
U_ADDER_5: IC73.4(D0)
U_ADDER_6: IC34.4(D0)
U_ADDER_7: IC35.4(D0)
U_ADDER_8: IC36.4(D0)
U_ADDER_9: IC37.4(D0)
U_ADDER_10: IC38.4(D0)
U_ADDER_11: IC40.4(D0)
U_ADDER_12: IC41.4(D0)
U_ADDER_13: IC53.1(S2) IC71.4(D0)
U_ADDR_MUX_1: IC42.3(A:O)
U_CF: IC126.5(2Q) IC155.11(2C1) IC167.3(1B)
U_DMA_0: IC186.14(D5)
U_DMA_1: IC160.14(D5)
U_DMA_2: IC159.14(D5)
U_DMA_3: IC142.14(D5)
U_DMA_4: IC129.14(D5)
U_DMA_5: IC73.14(D5)
U_DMA_6: IC34.14(D5)
U_DMA_7: IC35.14(D5)
U_DMA_8: IC36.14(D5)
U_DMA_9: IC37.14(D5)
U_DMA_10: IC38.14(D5)
U_DMA_11: IC40.14(D5)
U_DMA_12: IC41.14(D5)
U_DMA_13: IC71.14(D5)
U_FETCH_0: IC186.2(D2)
U_FETCH_1: IC160.2(D2)
U_FETCH_2: IC159.2(D2)
U_FETCH_3: IC142.2(D2)
U_FETCH_4: IC129.2(D2)
U_FETCH_5: IC73.2(D2)
U_FETCH_6: IC34.2(D2)
U_FETCH_7: IC35.2(D2)
U_FETCH_8: IC36.2(D2)
U_FETCH_9: IC37.2(D2)
U_FETCH_10: IC38.2(D2)
U_FETCH_11: IC40.2(D2)
U_FETCH_12: IC41.2(D2)
U_FETCH_13: IC71.2(D2)
U_FLAGS_REG_WRT: IC126.1(G)
U_INTERRUPT_0: IC186.1(D3)
U_INTERRUPT_1: IC160.1(D3)
U_INTERRUPT_2: IC159.1(D3)
U_INTERRUPT_3: IC142.1(D3)
U_INTERRUPT_4: IC129.1(D3)
U_INTERRUPT_5: IC73.1(D3)
U_INTERRUPT_6: IC34.1(D3)
U_INTERRUPT_7: IC35.1(D3)
U_INTERRUPT_8: IC36.1(D3)
U_INTERRUPT_9: IC37.1(D3)
U_INTERRUPT_10: IC38.1(D3)
U_INTERRUPT_11: IC40.1(D3)
U_INTERRUPT_12: IC41.1(D3)
U_INTERRUPT_13: IC71.1(D3)
U_OF: IC126.9(4Q) IC156.11(2C1)
U_OFFSET0: IC49.3(1B)
U_OFFSET1: IC49.6(2B)
U_OFFSET2: IC49.10(3B)
U_OFFSET3: IC49.13(4B)
U_OFFSET4: IC55.3(1B)
U_OFFSET5: IC55.6(2B)
U_OFFSET6: IC55.10(3B)
U_SF: IC126.6(3Q) IC156.5(1C1)
U_TRAP_0: IC186.15(D4)
U_TRAP_1: IC160.15(D4)
U_TRAP_2: IC159.15(D4)
U_TRAP_3: IC142.15(D4)
U_TRAP_4: IC129.15(D4)
U_TRAP_5: IC73.15(D4)
U_TRAP_6: IC34.15(D4)
U_TRAP_7: IC35.15(D4)
U_TRAP_8: IC36.15(D4)
U_TRAP_9: IC37.15(D4)
U_TRAP_10: IC38.15(D4)
U_TRAP_11: IC40.15(D4)
U_TRAP_12: IC41.15(D4)
U_TRAP_13: IC71.15(D4)
U_ZF: IC47.1(A:I0) IC126.2(1Q) IC127.2(A:I1) IC155.5(1C1)
U_ZF_IN_SRC: IC121.1(!A!/B)
UZF_AND_ALUZF: IC47.2(A:I1) IC119.3(B:I)
VCC: IC8.2(A:D) IC8.4(A:PRE) IC44.1(A:CLR) IC49.2(1A) IC56.5(1C1) IC163.2(A:D) IC163.4(A:PRE) IC164.2(A:D) IC164.4(A:PRE) IC168.2(A:D) IC168.4(A:PRE) IC174.2(A:D) IC174.4(A:PRE) IC187.2(A:D) IC187.4(A:PRE) IC188.2(A:D) IC188.4(A:PRE) IC204.4(A:PRE) IC221.2(A:D) IC221.4(A:PRE) IC222.6(G1) R1.2 R2.2 R3.2 R9.2
WR: IC69.7(B:Y2) RN4.15
XBUS0: IC2.18(Y1) IC9.18(Y1) IC25.9(B:Y1) IC27.9(B:Y1) IC103.18(Y1) IC104.18(Y1) IC105.9(B:Y1) IC107.9(B:Y1) IC109.9(B:Y1) IC111.9(B:Y1) IC113.18(Y1) IC114.18(Y1) IC116.18(Y1) IC117.18(Y1) IC122.18(Y1) IC125.18(Y1) IC140.18(Y1) IC145.18(Y1) IC154.18(Y1) IC181.18(A:Y1) IC210.18(Y1) IC244.9(B:Y1) IC245.18(Y1) RN1.1
XBUS1: IC2.17(Y2) IC9.17(Y2) IC25.7(B:Y2) IC27.7(B:Y2) IC105.7(B:Y2) IC107.7(B:Y2) IC109.7(B:Y2) IC111.7(B:Y2) IC113.17(Y2) IC114.17(Y2) IC116.17(Y2) IC117.17(Y2) IC122.17(Y2) IC125.17(Y2) IC145.17(Y2) IC154.17(Y2) IC181.16(A:Y2) IC245.17(Y2) RN1.2
XBUS2: IC2.16(Y3) IC9.16(Y3) IC25.5(B:Y3) IC27.5(B:Y3) IC105.5(B:Y3) IC107.5(B:Y3) IC109.5(B:Y3) IC111.5(B:Y3) IC113.16(Y3) IC114.16(Y3) IC116.16(Y3) IC117.16(Y3) IC122.16(Y3) IC125.16(Y3) IC145.16(Y3) IC154.16(Y3) IC181.14(A:Y3) IC245.16(Y3) RN1.3
XBUS3: IC2.15(Y4) IC9.15(Y4) IC25.3(B:Y4) IC27.3(B:Y4) IC105.3(B:Y4) IC107.3(B:Y4) IC109.3(B:Y4) IC111.3(B:Y4) IC113.15(Y4) IC114.15(Y4) IC116.15(Y4) IC117.15(Y4) IC122.15(Y4) IC125.15(Y4) IC145.15(Y4) IC154.15(Y4) IC181.12(A:Y4) IC244.3(B:Y4) IC245.15(Y4) RN1.4
XBUS4: IC24.9(B:Y1) IC26.9(B:Y1) IC106.9(B:Y1) IC108.9(B:Y1) IC110.9(B:Y1) IC112.9(B:Y1) IC116.14(Y5) IC125.14(Y5) IC154.14(Y5) IC176.18(A:Y1) IC245.14(Y5) IC247.9(B:Y1) RN1.5
XBUS5: IC24.7(B:Y2) IC26.7(B:Y2) IC106.7(B:Y2) IC108.7(B:Y2) IC110.7(B:Y2) IC112.7(B:Y2) IC116.13(Y6) IC125.13(Y6) IC154.13(Y6) IC176.16(A:Y2) IC245.13(Y6) RN1.6
XBUS6: IC24.5(B:Y3) IC26.5(B:Y3) IC106.5(B:Y3) IC108.5(B:Y3) IC110.5(B:Y3) IC112.5(B:Y3) IC113.12(Y7) IC114.12(Y7) IC115.12(Y7) IC116.12(Y7) IC125.12(Y7) IC154.12(Y7) IC176.14(A:Y3) IC245.12(Y7) RN1.7
XBUS7: IC2.11(Y8) IC3.11(Y8) IC9.11(Y8) IC24.3(B:Y4) IC26.3(B:Y4) IC80.4(B:I0) IC102.11(Y8) IC103.11(Y8) IC104.11(Y8) IC106.3(B:Y4) IC108.3(B:Y4) IC110.3(B:Y4) IC112.3(B:Y4) IC113.11(Y8) IC114.11(Y8) IC115.11(Y8) IC116.11(Y8) IC117.11(Y8) IC122.11(Y8) IC125.11(Y8) IC130.5(B:I1) IC140.11(Y8) IC145.11(Y8) IC146.11(Y8) IC154.11(Y8) IC176.12(A:Y4) IC210.11(Y8) IC245.11(Y8) IC247.3(B:Y4) RN1.8
XBUS8: IC146.18(Y1)
XBUS9: IC146.17(Y2)
XBUS10: IC146.16(Y3)
XBUS11: IC146.15(Y4)
XBUS12: IC171.18(Y1) IC215.18(Y1)
XBUS13: IC171.11(Y8) IC215.11(Y8)
XBUS14: IC259.18(Y1) IC260.18(Y1)
XBUS15: IC259.11(Y8) IC260.11(Y8)
XBUS16: IC89.18(A:Y1) IC91.18(A:Y1)
XBUS17: IC89.16(A:Y2) IC91.16(A:Y2)
XBUS18: IC89.14(A:Y3) IC91.14(A:Y3)
XBUS19: IC89.12(A:Y4) IC91.12(A:Y4)
XBUS20: IC90.18(A:Y1) IC92.18(A:Y1)
XBUS21: IC90.16(A:Y2) IC92.16(A:Y2)
XBUS22: IC90.14(A:Y3) IC92.14(A:Y3)
XBUS23: IC90.12(A:Y4) IC92.12(A:Y4)
XBUS24: IC14.1(B0) RN2.1
XBUS25: IC14.22(B1) RN2.2
XBUS26: IC14.20(B2) RN2.3
XBUS27: IC14.18(B3) RN2.4
XBUS28: IC11.12(A:Y4) IC15.1(B0) RN2.5
XBUS29: IC11.14(A:Y3) IC15.22(B1) RN2.6
XBUS30: IC11.16(A:Y2) IC15.20(B2) RN2.7
XBUS31: IC11.18(A:Y1) IC15.18(B3) RN2.8
XBUS32: IC102.18(Y1)
XBUS33: IC102.17(Y2)
XBUS34: IC102.16(Y3)
XBUS35: IC102.15(Y4)
XBUS36: IC263.18(Y1) IC264.18(Y1)
XBUS37: IC263.11(Y8) IC264.11(Y8)
XBUS40: IC3.18(Y1)
XBUS41: IC3.17(Y2)
XBUS42: IC3.16(Y3)
XBUS43: IC3.15(Y4)
XBUS48: IC115.18(Y1)
XBUS49: IC115.17(Y2)
XBUS50: IC115.16(Y3)
XBUS51: IC115.15(Y4)
XBUS56: IC15.19(A3) RN3.1
XBUS57: IC15.21(A2) RN3.2
XBUS58: IC15.23(A1) RN3.3
XBUS59: IC15.2(A0) RN3.4
XBUS60: IC14.19(A3) RN3.5
XBUS61: IC14.21(A2) RN3.6
XBUS62: IC14.23(A1) RN3.7
XBUS63: IC14.2(A0) RN3.8
YBUS0: IC19.18(Y1) IC182.18(A:Y1)
YBUS1: IC19.17(Y2) IC182.16(A:Y2)
YBUS2: IC19.16(Y3) IC182.14(A:Y3)
YBUS3: IC19.15(Y4) IC182.12(A:Y4)
YBUS4: IC19.14(Y5) IC183.18(A:Y1)
YBUS5: IC183.16(A:Y2)
YBUS6: IC183.14(A:Y3)
YBUS7: IC19.11(Y8) IC130.4(B:I0) IC183.12(A:Y4)
YBUS16: IC211.18(A:Y1) IC213.18(A:Y1)
YBUS17: IC211.16(A:Y2) IC213.16(A:Y2)
YBUS18: IC211.14(A:Y3) IC213.14(A:Y3)
YBUS19: IC211.12(A:Y4) IC213.12(A:Y4)
YBUS20: IC212.18(A:Y1) IC214.18(A:Y1)
YBUS21: IC212.16(A:Y2) IC214.16(A:Y2)
YBUS22: IC212.14(A:Y3) IC214.14(A:Y3)
YBUS23: IC212.12(A:Y4) IC214.12(A:Y4)
YBUS40: IC229.18(A:Y1) IC231.18(A:Y1)
YBUS41: IC229.16(A:Y2) IC231.16(A:Y2)
YBUS42: IC229.14(A:Y3) IC231.14(A:Y3)
YBUS43: IC229.12(A:Y4) IC231.12(A:Y4)
YBUS44: IC230.18(A:Y1) IC232.18(A:Y1)
YBUS45: IC230.16(A:Y2) IC232.16(A:Y2)
YBUS46: IC230.14(A:Y3) IC232.14(A:Y3)
YBUS47: IC230.12(A:Y4) IC232.12(A:Y4)
YBUS48: IC235.18(A:Y1) IC237.18(A:Y1)
YBUS49: IC235.16(A:Y2) IC237.16(A:Y2)
YBUS50: IC235.14(A:Y3) IC237.14(A:Y3)
YBUS51: IC235.12(A:Y4) IC237.12(A:Y4)
YBUS52: IC236.18(A:Y1) IC238.18(A:Y1)
YBUS53: IC236.16(A:Y2) IC238.16(A:Y2)
YBUS54: IC236.14(A:Y3) IC238.14(A:Y3)
YBUS55: IC236.12(A:Y4) IC238.12(A:Y4)
ZBUFF0_16: IC86.3(1D) IC88.3(1D)
ZBUFF0_17: IC86.4(2D) IC88.4(2D)
ZBUFF0_18: IC86.7(3D) IC88.7(3D)
ZBUFF0_19: IC86.8(4D) IC88.8(4D)
ZBUFF0_20: IC86.13(5D) IC88.13(5D)
ZBUFF0_21: IC88.14(6D)
ZBUFF0_22: IC86.14(6D) IC86.17(7D) IC88.17(7D)
ZBUFF0_23: IC86.18(8D) IC88.18(8D)
ZBUFF0_24: IC16.3(1D) IC17.3(1D)
ZBUFF0_25: IC16.4(2D) IC17.4(2D)
ZBUFF0_26: IC16.7(3D) IC17.7(3D)
ZBUFF0_27: IC16.8(4D) IC17.8(4D)
ZBUFF0_28: IC16.13(5D) IC17.13(5D)
ZBUFF0_29: IC16.14(6D) IC17.14(6D)
ZBUFF0_30: IC16.17(7D) IC17.17(7D)
ZBUFF0_31: IC16.18(8D) IC17.18(8D)
ZBUFF0_56: IC233.3(1D) IC234.3(1D)
ZBUFF0_57: IC233.4(2D) IC234.4(2D)
ZBUFF0_58: IC233.7(3D) IC234.7(3D)
ZBUFF0_59: IC233.8(4D) IC234.8(4D)
ZBUFF0_60: IC233.13(5D) IC234.13(5D)
ZBUFF0_61: IC233.14(6D) IC234.14(6D)
ZBUFF0_62: IC233.17(7D) IC234.17(7D)
ZBUFF0_63: IC233.18(8D) IC234.18(8D)
ZBUFF0_64: IC239.3(1D) IC240.3(1D)
ZBUFF0_65: IC239.4(2D) IC240.4(2D)
ZBUFF0_66: IC239.7(3D) IC240.7(3D)
ZBUFF0_67: IC239.8(4D) IC240.8(4D)
ZBUFF0_68: IC239.13(5D) IC240.13(5D)
ZBUFF0_69: IC239.14(6D) IC240.14(6D)
ZBUFF0_70: IC239.17(7D) IC240.17(7D)
ZBUFF0_71: IC239.18(8D) IC240.18(8D)
ZBUFF1_0: IC4.3(1D) IC5.3(1D) IC98.3(1D) IC99.3(1D)
ZBUFF1_1: IC4.4(2D) IC5.4(2D) IC98.4(2D) IC99.4(2D)
ZBUFF1_2: IC4.7(3D) IC5.7(3D) IC98.7(3D) IC99.7(3D)
ZBUFF1_3: IC4.8(4D) IC5.8(4D) IC98.8(4D) IC99.8(4D)
ZBUFF1_4: IC4.13(5D) IC5.13(5D) IC98.13(5D) IC99.13(5D)
ZBUFF1_5: IC4.14(6D) IC5.14(6D) IC98.14(6D) IC99.14(6D)
ZBUFF1_6: IC4.17(7D) IC5.17(7D) IC98.17(7D) IC99.17(7D)
ZBUFF1_7: IC4.18(8D) IC5.18(8D) IC98.18(8D) IC99.18(8D)
ZBUFF1_8: IC173.3(1D) IC205.3(1D)
ZBUFF1_9: IC173.4(2D) IC205.4(2D)
ZBUFF1_10: IC173.7(3D) IC205.7(3D)
ZBUFF1_11: IC173.8(4D) IC205.8(4D)
ZBUFF1_12: IC173.13(5D) IC205.13(5D)
ZBUFF1_13: IC173.14(6D) IC205.14(6D)
ZBUFF1_14: IC173.17(7D) IC205.17(7D)
ZBUFF1_15: IC173.18(8D) IC205.18(8D)
ZBUFF1_16: IC165.3(1D) IC166.3(1D)
ZBUFF1_17: IC165.4(2D) IC166.4(2D)
ZBUFF1_18: IC165.7(3D) IC166.7(3D)
ZBUFF1_19: IC165.8(4D) IC166.8(4D)
ZBUFF1_20: IC165.13(5D) IC166.13(5D)
ZBUFF1_21: IC165.14(6D) IC166.14(6D)
ZBUFF1_22: IC165.17(7D) IC166.17(7D)
ZBUFF1_23: IC165.18(8D) IC166.18(8D)
ZBUFF1_24: IC217.3(1D) IC246.3(1D)
ZBUFF1_25: IC217.4(2D) IC246.4(2D)
ZBUFF1_26: IC217.7(3D) IC246.7(3D)
ZBUFF1_27: IC217.8(4D) IC246.8(4D)
ZBUFF1_28: IC217.13(5D) IC246.13(5D)
ZBUFF1_29: IC217.14(6D) IC246.14(6D)
ZBUFF1_30: IC217.17(7D) IC246.17(7D)
ZBUFF1_31: IC217.18(8D) IC246.18(8D)
ZBUFF1_32: IC261.3(1D) IC262.3(1D)
ZBUFF1_33: IC261.4(2D) IC262.4(2D)
ZBUFF1_34: IC261.7(3D) IC262.7(3D)
ZBUFF1_35: IC261.8(4D) IC262.8(4D)
ZBUFF1_36: IC261.13(5D) IC262.13(5D)
ZBUFF1_37: IC261.14(6D) IC262.14(6D)
ZBUFF1_38: IC261.17(7D) IC262.17(7D)
ZBUFF1_39: IC261.18(8D) IC262.18(8D)
ZBUFF2_0: IC1.3(1D) IC23.14(4A) IC100.3(1D) IC101.3(1D)
ZBUFF2_1: IC1.4(2D) IC23.11(3A) IC100.4(2D) IC101.4(2D)
ZBUFF2_2: IC1.7(3D) IC23.5(2A) IC100.7(3D) IC101.7(3D)
ZBUFF2_3: IC1.8(4D) IC23.2(1A) IC100.8(4D) IC101.8(4D)
ZBUFF2_4: IC1.13(5D) IC22.14(4A) IC100.13(5D) IC101.13(5D)
ZBUFF2_5: IC1.14(6D) IC22.11(3A) IC100.14(6D) IC101.14(6D)
ZBUFF2_6: IC1.17(7D) IC22.5(2A) IC100.17(7D) IC101.17(7D)
ZBUFF2_7: IC22.2(1A) IC100.18(8D) IC101.18(8D)
ZBUFF2_16: IC123.3(1D)
ZBUFF2_17: IC123.4(2D)
ZBUFF2_18: IC123.7(3D)
ZBUFF2_19: IC123.8(4D)
ZBUFF2_20: IC123.13(5D)
ZBUFF2_21: IC123.14(6D)
ZBUFF2_22: IC123.17(7D)
ZBUFF2_23: IC153.3(1D)
ZBUFF2_24: IC153.4(2D)
ZBUFF2_25: IC153.7(3D)
ZBUFF2_26: IC153.8(4D)
ZBUFF2_27: IC153.13(5D)
ZBUFF2_28: IC153.14(6D)
ZBUFF2_29: IC153.17(7D)
ZBUFF2_30: IC153.18(8D)
ZBUFF2_31: IC185.3(1D)
ZBUFF2_32: IC185.4(2D)
ZBUFF2_33: IC185.7(3D)
ZBUFF2_34: IC185.8(4D)
ZBUFF2_35: IC185.13(5D)
ZBUFF2_36: IC185.14(6D)
ZBUFF2_37: IC185.17(7D)
ZBUFF2_38: IC185.18(8D)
